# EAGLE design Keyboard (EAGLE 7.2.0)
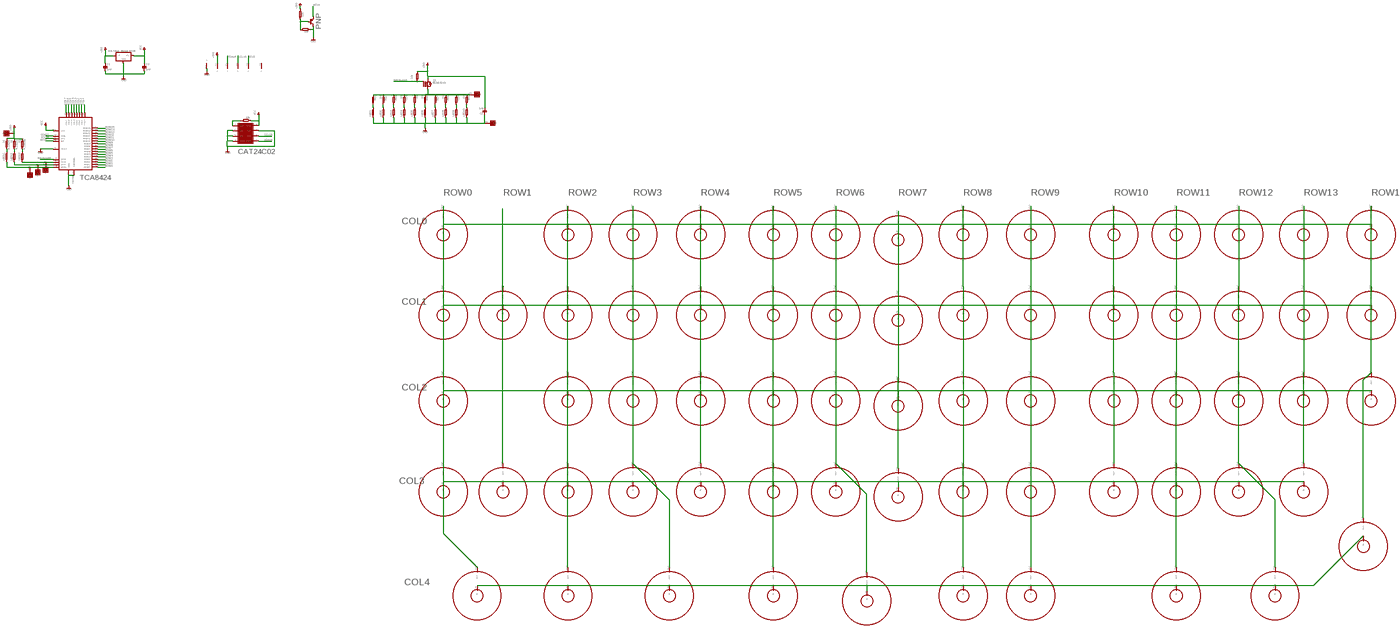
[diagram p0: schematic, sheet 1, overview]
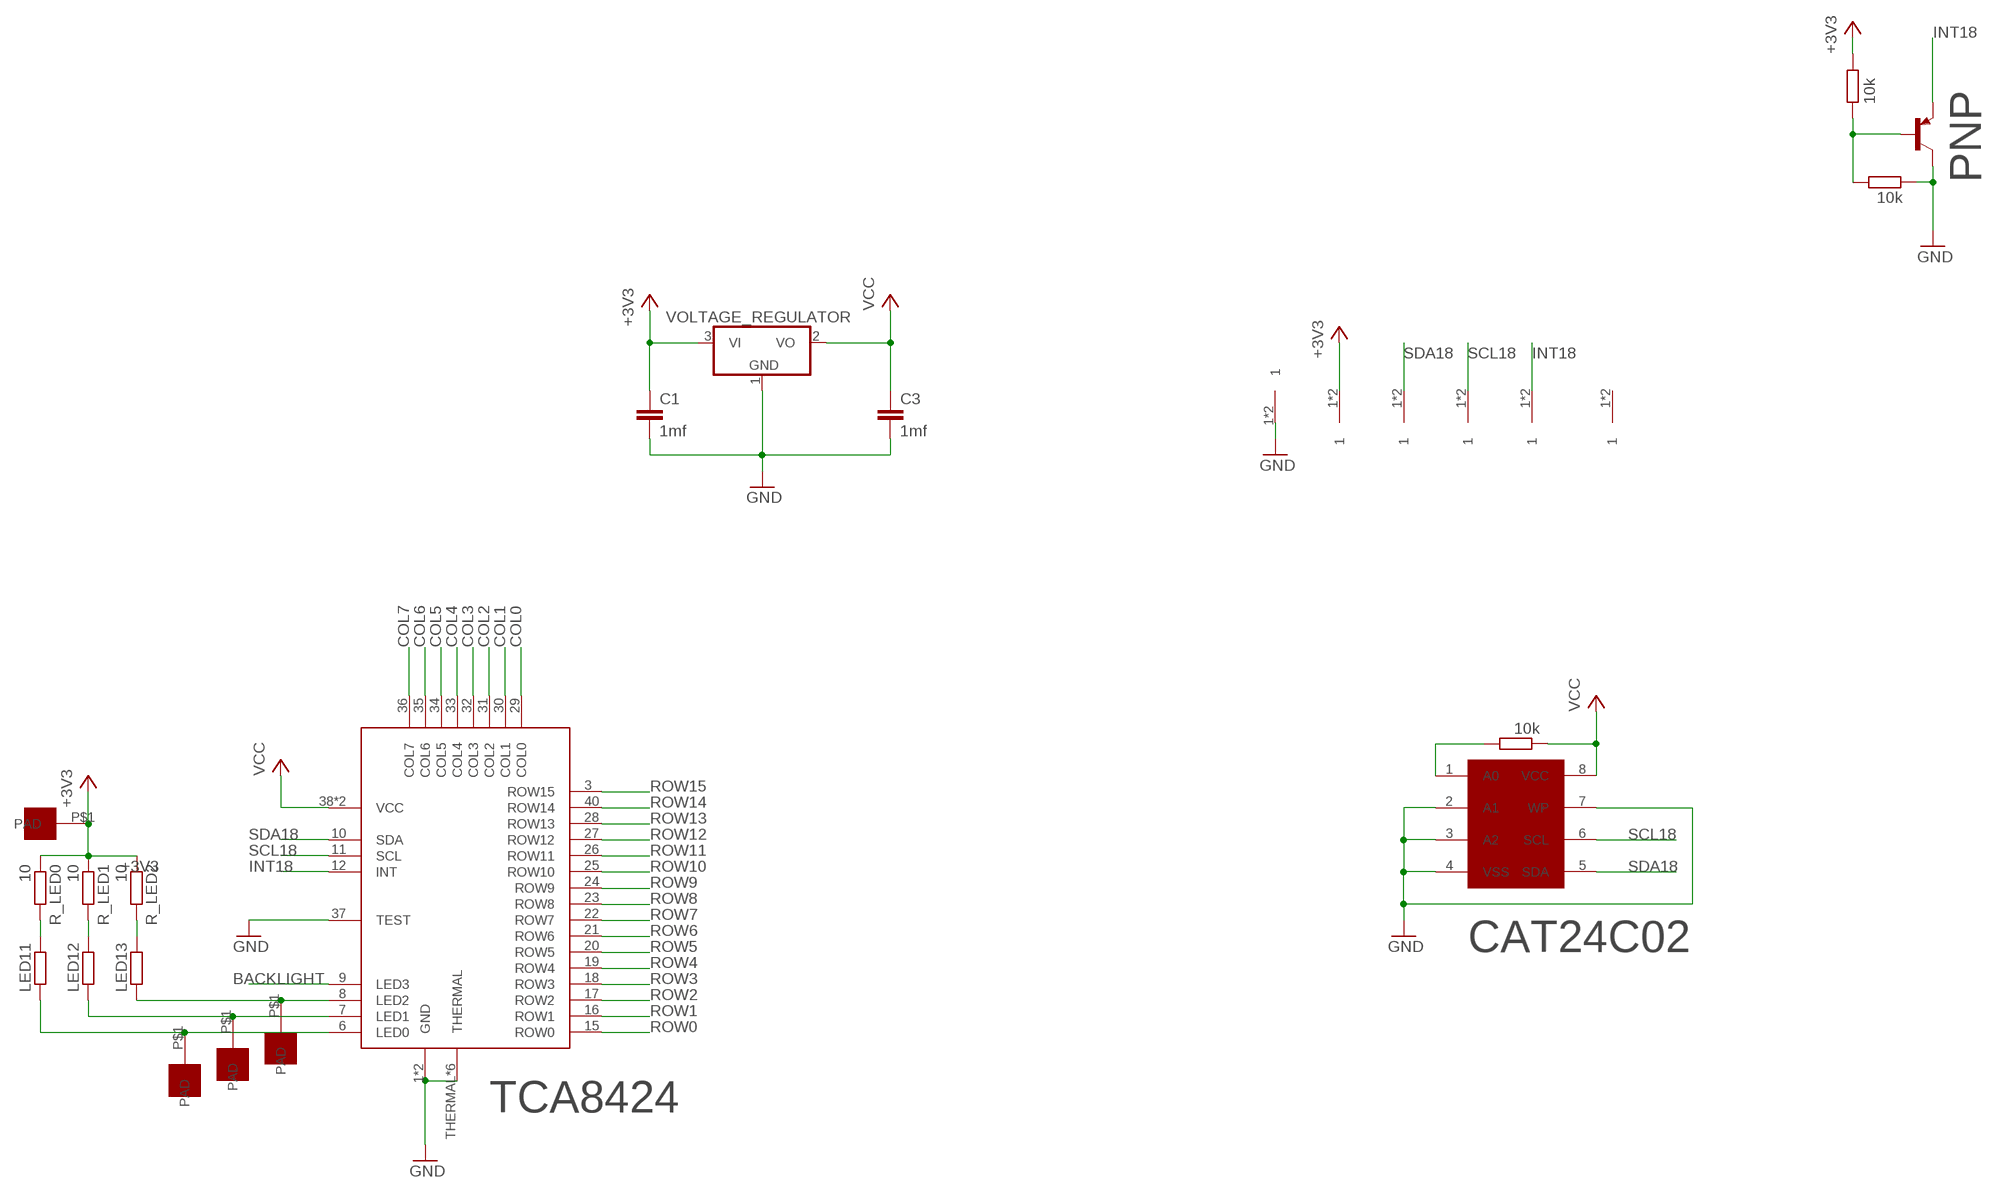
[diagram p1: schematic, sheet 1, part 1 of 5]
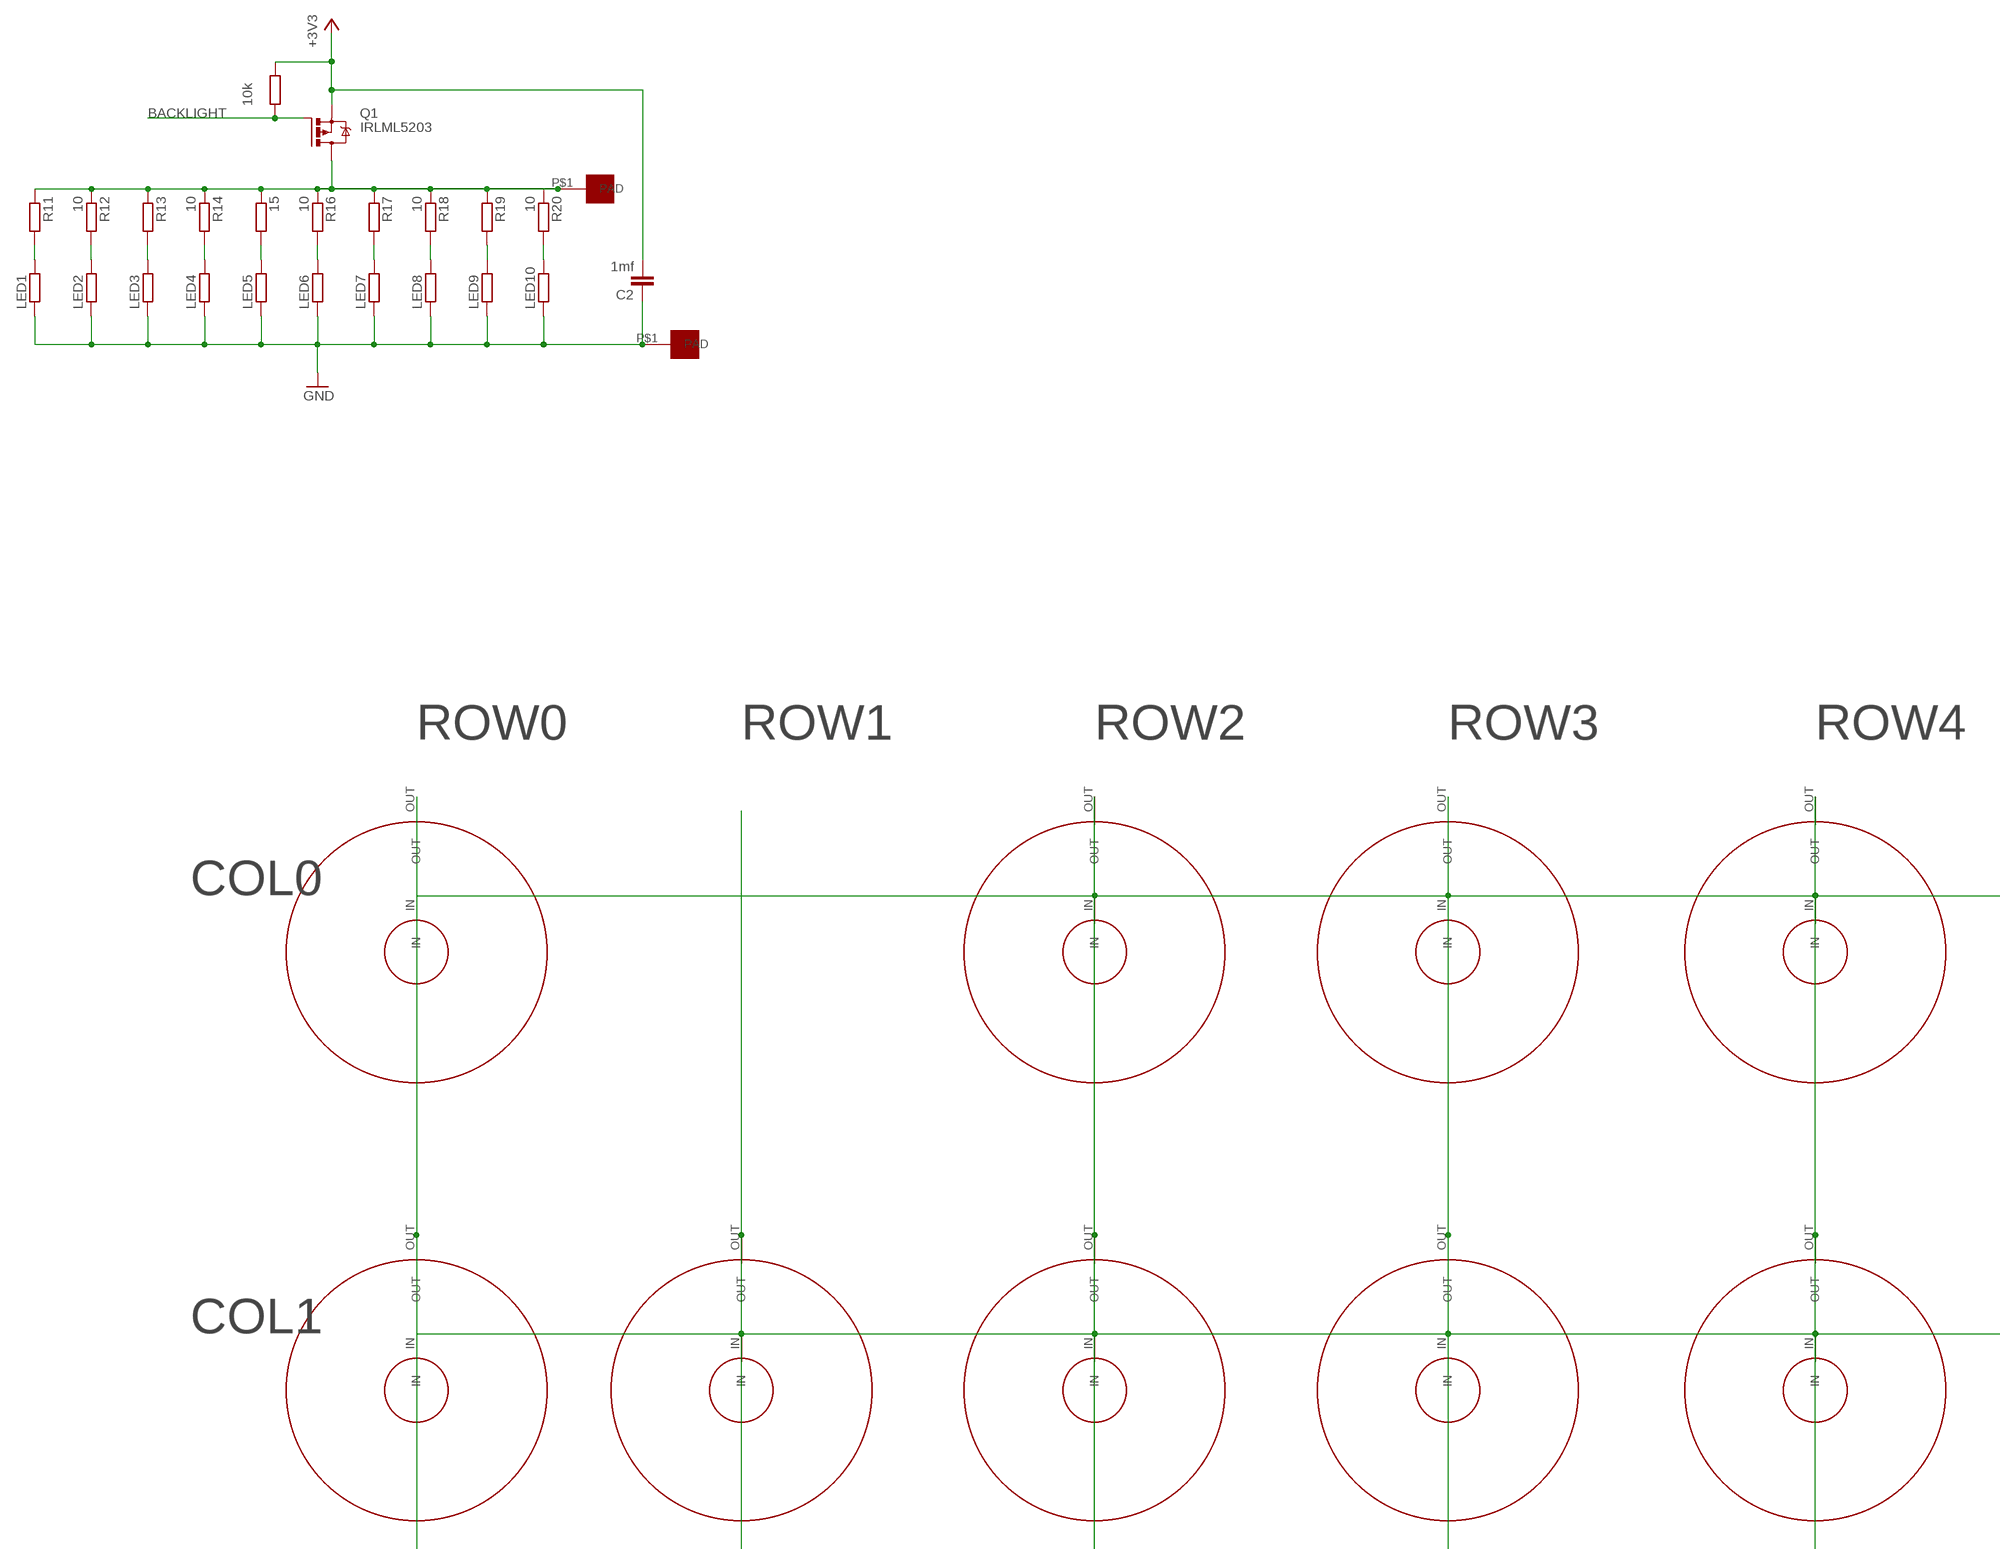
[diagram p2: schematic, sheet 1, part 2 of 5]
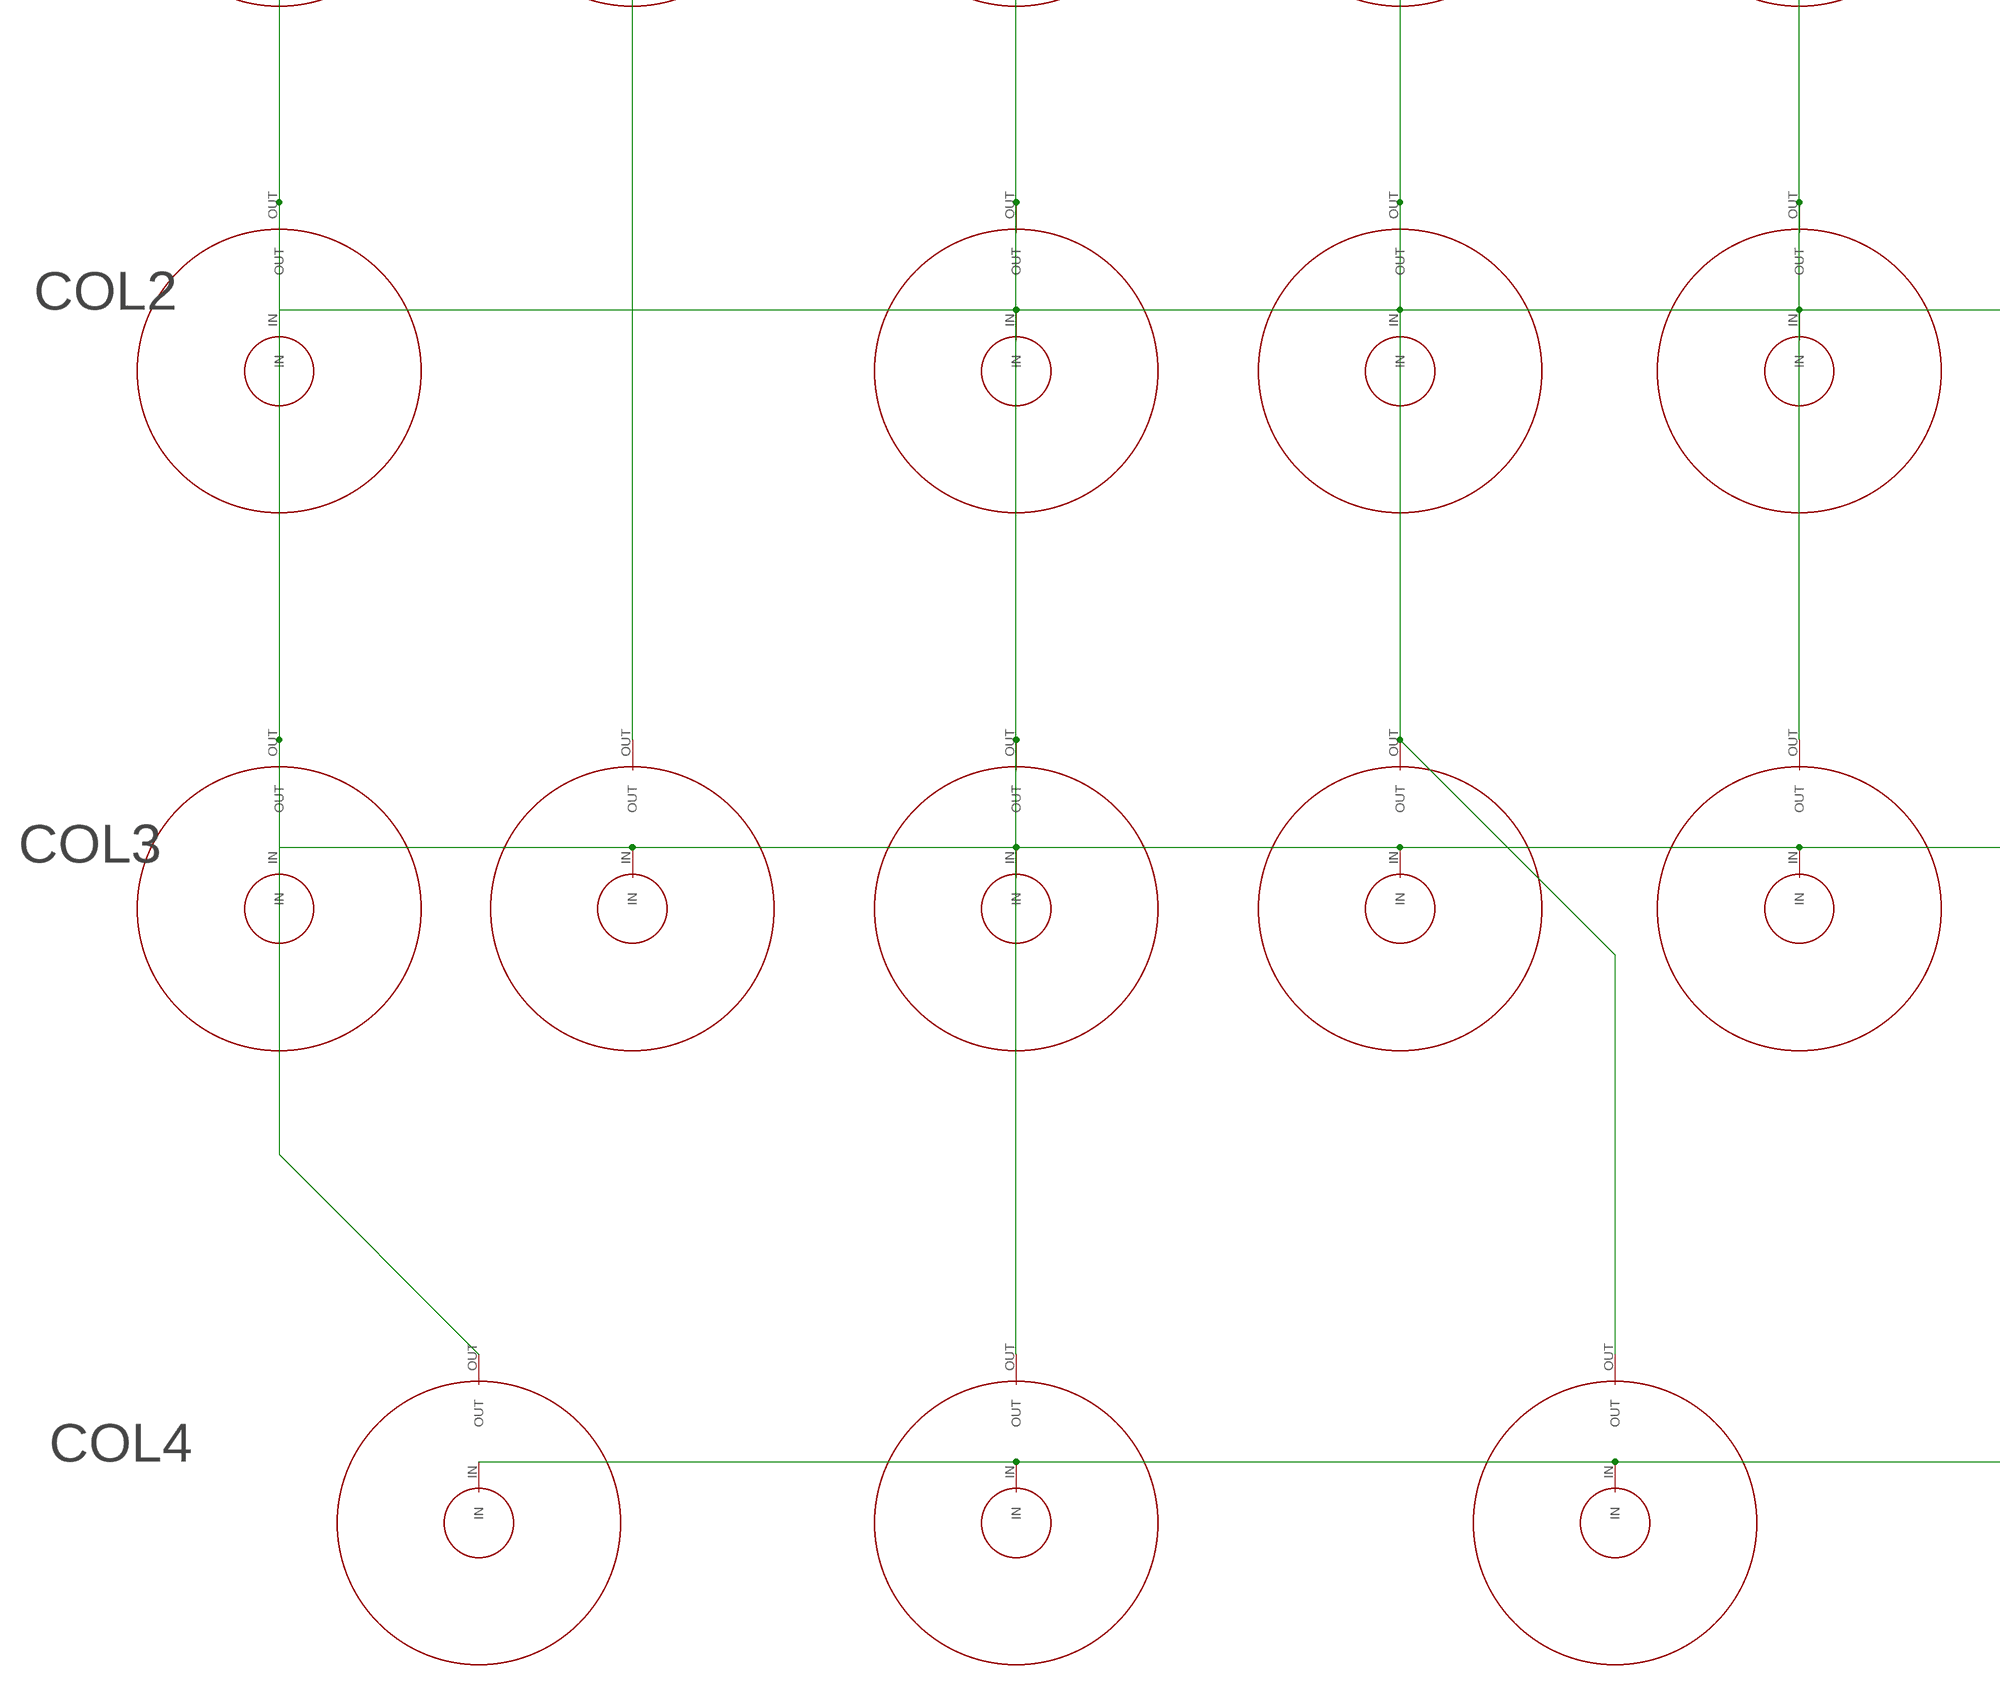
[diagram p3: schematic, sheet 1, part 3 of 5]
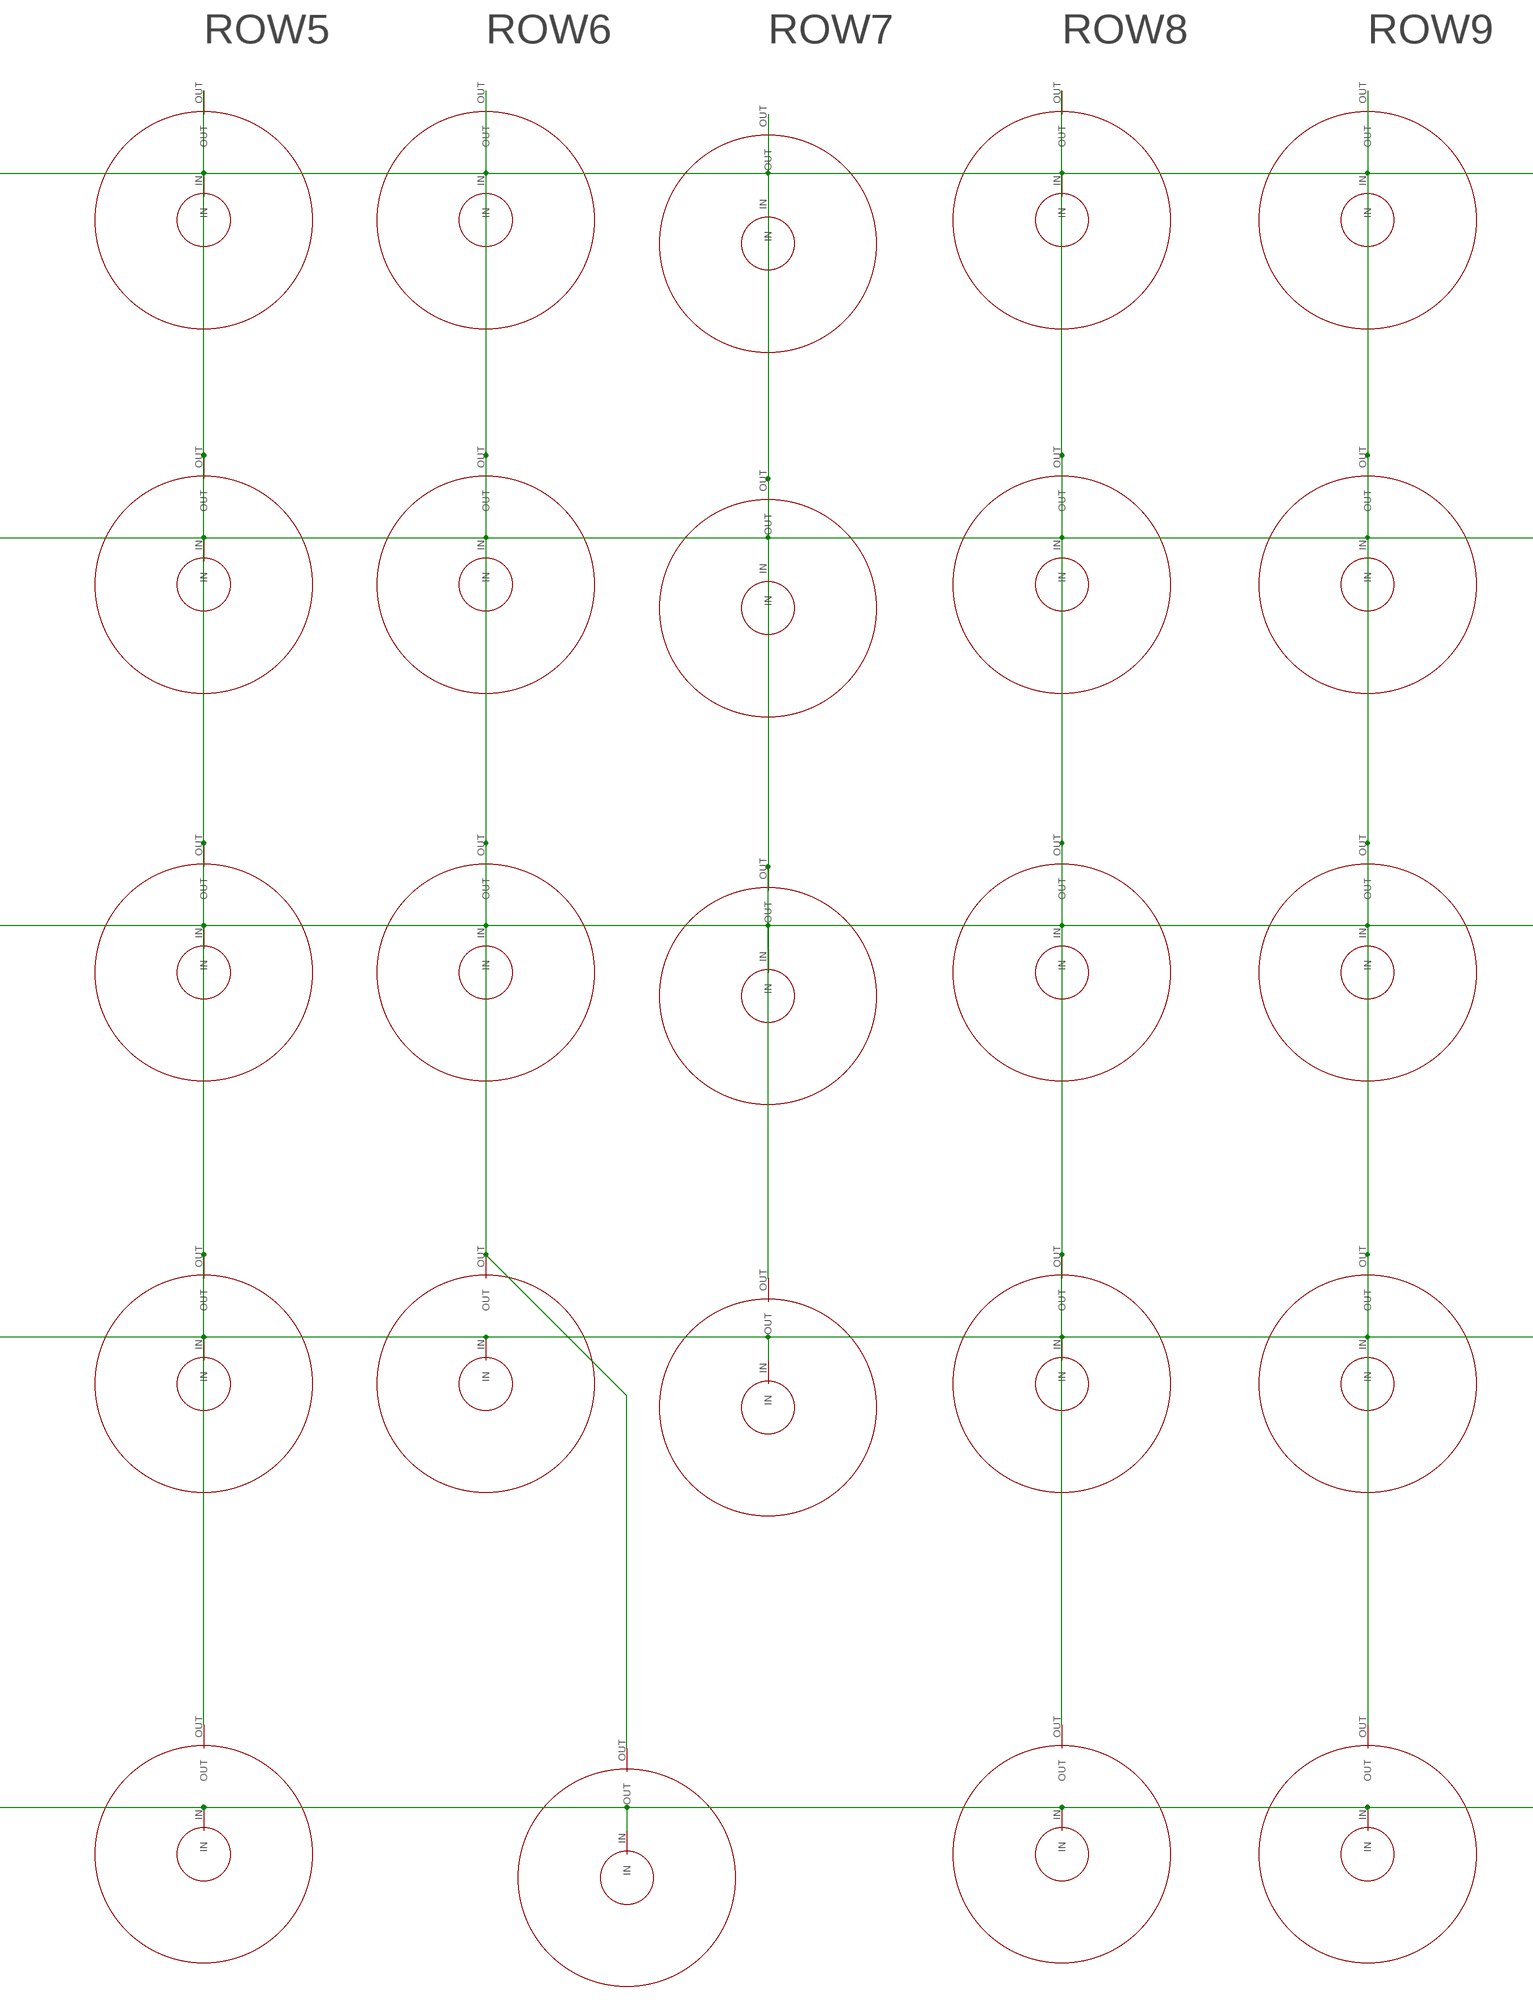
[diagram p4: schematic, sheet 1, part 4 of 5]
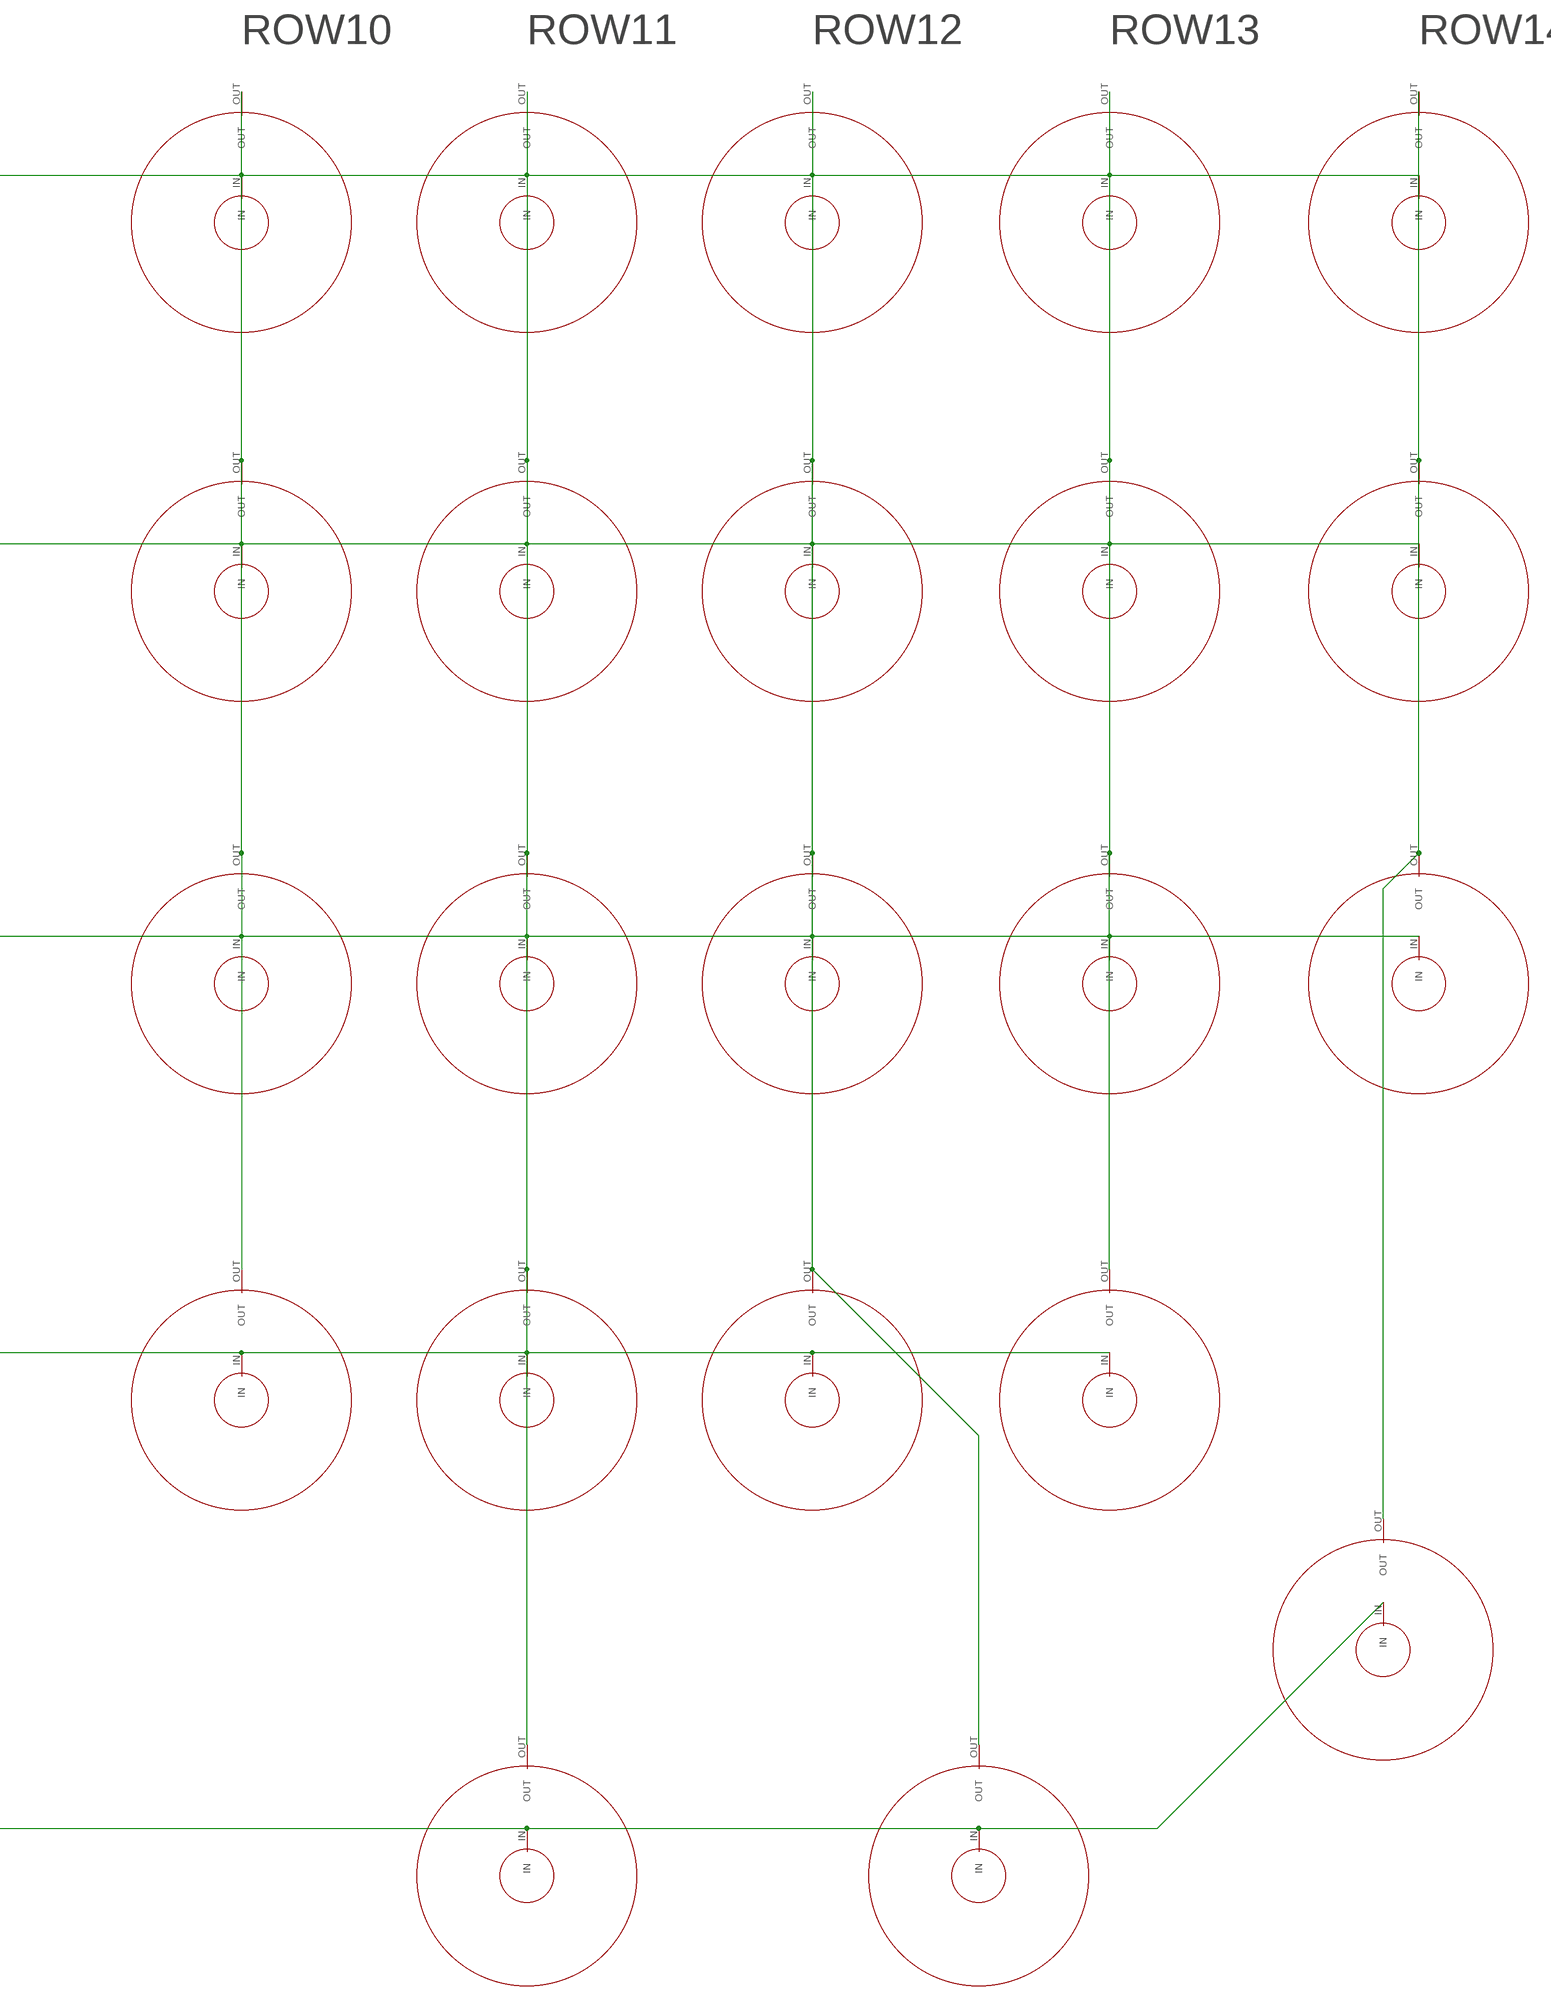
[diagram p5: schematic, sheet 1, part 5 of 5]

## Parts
15  R-EU_R0603  [R0603]
+  PAD  [PAD]
BL_PULLUP  10k  R-EU_R0603  [R0603]
C1  1mf  C-EUC0603  [C0603]
C2  1mf  C-EUC0603  [C0603]
C3  1mf  C-EUC0603  [C0603]
LED1  R-EU_R0402  [R0402]
LED2  R-EU_R0402  [R0402]
LED3  R-EU_R0402  [R0402]
LED4  R-EU_R0402  [R0402]
LED5  R-EU_R0402  [R0402]
LED6  R-EU_R0402  [R0402]
LED7  R-EU_R0402  [R0402]
LED8  R-EU_R0402  [R0402]
LED9  R-EU_R0402  [R0402]
LED10  R-EU_R0402  [R0402]
LED11  R-EU_R0402  [R0402]
LED12  R-EU_R0402  [R0402]
LED13  R-EU_R0402  [R0402]
PNP_DOWN  10k  R-EU_R0603  [R0603]
PNP_DOWN1  10k  R-EU_R0603  [R0603]
PNP_UP  10k  R-EU_R0603  [R0603]
Q1  IRLML5203  [MICRO3]
Q2  MMBTA56-SOT23  [SOT23]
R11  R-EU_R0603  [R0603]
R12  10  R-EU_R0603  [R0603]
R13  R-EU_R0603  [R0603]
R14  10  R-EU_R0603  [R0603]
R16  10  R-EU_R0603  [R0603]
R17  R-EU_R0603  [R0603]
R18  10  R-EU_R0603  [R0603]
R19  R-EU_R0603  [R0603]
R20  10  R-EU_R0603  [R0603]
R_LED0  10  R-EU_R0603  [R0603]
R_LED1  10  R-EU_R0603  [R0603]
R_LED2  10  R-EU_R0603  [R0603]
U$1  CAT24  [CAT24]
U$2  TCA8424  [QFN40]
U$3  BOTTOM_POGO  [POGO]
U$4  BOTTOM_POGO  [POGO]
U$5  BOTTOM_POGO  [POGO]
U$6  BOTTOM_POGO  [POGO]
U$7  BOTTOM_POGO  [POGO]
U$8  BOTTOM_POGO  [POGO]
U$9  DOME  [4MM]
U$11  DOME  [4MM]
U$12  DOME  [4MM]
U$13  DOME  [4MM]
U$14  DOME  [4MM]
U$15  DOME  [4MM]
U$16  DOME  [4MM]
U$17  DOME  [4MM]
U$18  DOME  [4MM]
U$19  DOME  [4MM]
U$20  DOME  [4MM]
U$21  DOME  [4MM]
U$22  DOME  [4MM]
U$23  DOME  [4MM]
U$24  DOME  [4MM]
U$25  DOME  [4MM]
U$26  DOME  [4MM]
U$27  DOME  [4MM]
U$28  DOME  [4MM]
U$29  DOME  [4MM]
U$30  DOME  [4MM]
U$31  DOME  [4MM]
U$32  DOME  [4MM]
U$33  DOME  [4MM]
U$34  DOME  [4MM]
U$35  DOME  [4MM]
U$36  DOME  [4MM]
U$37  DOME  [4MM]
U$38  DOME  [4MM]
U$39  DOME  [4MM]
U$40  DOME  [4MM]
U$41  DOME  [4MM]
U$42  DOME  [4MM]
U$43  DOME  [4MM]
U$44  DOME  [4MM]
U$45  DOME  [4MM]
U$46  DOME  [4MM]
U$47  DOME  [4MM]
U$48  DOME  [4MM]
U$49  DOME  [4MM]
U$50  DOME  [4MM]
U$51  DOME  [4MM]
U$52  DOME  [4MM]
U$53  PAD  [PAD]
U$54  DOME  [4MM]
U$55  DOME  [4MM]
U$56  DOME  [4MM]
U$57  DOME  [4MM]
U$58  DOME  [4MM]
U$59  DOME  [4MM]
U$60  DOME  [4MM]
U$61  DOME  [4MM]
U$62  DOME  [4MM]
U$63  DOME  [4MM]
U$64  DOME  [4MM]
U$65  DOME  [4MM]
U$66  DOME  [4MM]
U$67  DOME  [4MM]
U$68  DOME  [4MM]
U$69  DOME  [4MM]
U$70  DOME  [4MM]
U$71  PAD  [PAD]
U$72  DOME  [4MM]
U$73  DOME  [4MM]
U$74  PAD  [PAD]
U$75  DOME  [4MM]
U$76  DOME  [4MM]
U$77  DOME  [4MM]
U$78  PAD  [PAD]
U$79  DOME  [4MM]
U$80  PAD  [PAD]
U$81  DOME  [4MM]
VOLTAGE_REGULATOR  MCP1703CB  [SOT23]

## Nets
+3V3: +.P$1(PAD) BL_PULLUP.1 C1.1 C2.2 PNP_UP.1 Q1.2(S) R_LED0.1 R_LED1.1 R_LED2.1 U$4.1 U$4.P$2 VOLTAGE_REGULATOR.3(VI)
BACKLIGHT: BL_PULLUP.2 Q1.1(G) U$2.9(LED3)
COL0: U$2.29(COL0) U$9.IN U$11.IN U$12.IN U$13.IN U$14.IN U$15.IN U$16.IN U$17.IN U$18.IN U$19.IN U$20.IN U$21.IN U$22.IN U$23.IN
COL1: U$2.30(COL1) U$24.IN U$25.IN U$26.IN U$27.IN U$28.IN U$29.IN U$30.IN U$31.IN U$32.IN U$33.IN U$34.IN U$35.IN U$36.IN U$37.IN U$38.IN
COL2: U$2.31(COL2) U$39.IN U$40.IN U$41.IN U$42.IN U$43.IN U$44.IN U$45.IN U$46.IN U$47.IN U$48.IN U$49.IN U$50.IN U$51.IN U$52.IN
COL3: U$2.32(COL3) U$54.IN U$55.IN U$56.IN U$57.IN U$58.IN U$59.IN U$60.IN U$61.IN U$62.IN U$63.IN U$64.IN U$65.IN U$66.IN U$68.IN
COL4: U$2.33(COL4) U$67.IN U$69.IN U$70.IN U$72.IN U$73.IN U$75.IN U$76.IN U$77.IN U$79.IN U$81.IN
COL5: U$2.34(COL5)
COL6: U$2.35(COL6)
COL7: U$2.36(COL7)
DRAIN: 15.1 Q1.3(D) R11.1 R12.1 R13.1 R14.1 R16.1 R17.1 R18.1 R19.1 R20.1 U$78.P$1(PAD)
GND: C1.2 C2.1 C3.2 LED1.1 LED2.1 LED3.1 LED4.1 LED5.1 LED6.1 LED7.1 LED8.1 LED9.1 LED10.1 PNP_DOWN.2 Q2.3(C) U$1.2(A1) U$1.3(A2) U$1.4(VSS) U$1.7(WP) U$2.1(GND) U$2.4(GND) U$2.37(TEST) U$2.THERMAL U$2.VIA1(THERMAL) U$2.VIA2(THERMAL) U$2.VIA3(THERMAL) U$2.VIA4(THERMAL) U$2.VIA5(THERMAL) U$3.1 U$3.P$2 U$80.P$1(PAD) VOLTAGE_REGULATOR.1(GND)
INT18: Q2.2(E) U$2.12(INT) U$7.1 U$7.P$2
LED_GROUND0: LED11.2 R_LED0.2
LED_GROUND1: LED12.2 R_LED1.2
LED_GROUND2: LED13.2 R_LED2.2
N$1: LED1.2 R11.2
N$2: LED2.2 R12.2
N$3: LED3.2 R13.2
N$4: LED4.2 R14.2
N$6: 15.2 LED5.2
N$7: LED6.2 R16.2
N$8: LED7.2 R17.2
N$9: LED8.2 R18.2
N$10: LED9.2 R19.2
N$11: LED10.2 R20.2
N$13: PNP_DOWN.1 PNP_UP.2 Q2.1(B)
N$14: LED12.1 U$2.7(LED1) U$71.P$1(PAD)
N$15: LED11.1 U$2.6(LED0) U$53.P$1(PAD)
N$16: LED13.1 U$2.8(LED2) U$74.P$1(PAD)
N$17: PNP_DOWN1.2 U$1.1(A0)
ROW0: U$2.15(ROW0) U$9.OUT U$24.OUT U$39.OUT U$54.OUT U$69.OUT
ROW1: U$2.16(ROW1) U$38.OUT U$68.OUT
ROW2: U$2.17(ROW2) U$11.OUT U$25.OUT U$40.OUT U$55.OUT U$70.OUT
ROW3: U$2.18(ROW3) U$12.OUT U$26.OUT U$41.OUT U$56.OUT U$72.OUT
ROW4: U$2.19(ROW4) U$13.OUT U$27.OUT U$42.OUT U$57.OUT
ROW5: U$2.20(ROW5) U$14.OUT U$28.OUT U$43.OUT U$58.OUT U$73.OUT
ROW6: U$2.21(ROW6) U$15.OUT U$29.OUT U$44.OUT U$59.OUT U$75.OUT
ROW7: U$2.22(ROW7) U$16.OUT U$30.OUT U$45.OUT U$60.OUT
ROW8: U$2.23(ROW8) U$17.OUT U$31.OUT U$46.OUT U$61.OUT U$76.OUT
ROW9: U$2.24(ROW9) U$18.OUT U$32.OUT U$47.OUT U$62.OUT U$77.OUT
ROW10: U$2.25(ROW10) U$19.OUT U$33.OUT U$48.OUT U$63.OUT
ROW11: U$2.26(ROW11) U$20.OUT U$34.OUT U$49.OUT U$64.OUT U$79.OUT
ROW12: U$2.27(ROW12) U$21.OUT U$35.OUT U$50.OUT U$65.OUT U$81.OUT
ROW13: U$2.28(ROW13) U$22.OUT U$36.OUT U$51.OUT U$66.OUT
ROW14: U$2.40(ROW14) U$23.OUT U$37.OUT U$52.OUT U$67.OUT
ROW15: U$2.3(ROW15)
SCL18: U$1.6(SCL) U$2.11(SCL) U$6.1 U$6.P$2
SDA18: U$1.5(SDA) U$2.10(SDA) U$5.1 U$5.P$2
VCC: C3.1 PNP_DOWN1.1 U$1.8(VCC) U$2.38(VCC) U$2.39(VCC) VOLTAGE_REGULATOR.2(VO)
Unconnected: U$8.1 U$8.P$2

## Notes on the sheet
- PNP
- CAT24C02
- TCA8424

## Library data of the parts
15 BL_PULLUP LED1-LED13 PNP_DOWN PNP_DOWN1 PNP_UP R11-R14 R16-R20 R_LED0 R_LED1 R_LED2 = rcl:R-EU_: RESISTOR, European symbol
+ U$53 U$71 U$74 U$78 U$80 = PAD:PAD
C1-C3 = rcl:C-EU: CAPACITOR, European symbol
Q1 = transistor-power:IRLML5203: HEXFET P-Channel Power MOSFET
Q2 = transistor-pnp:*-?: PNP Transistor
U$1 = cat24:CAT24
U$2 = TCA8424:TCA8424
U$3-U$8 = bottom_pogo:BOTTOM_POGO
U$9 U$11-U$52 U$54-U$70 U$72 U$73 U$75-U$77 U$79 U$81 = DOME:DOME
VOLTAGE_REGULATOR = linear:MCP1703: 250 mA, 16V, Low Quiescent Current LDO Regulator Source: http://ww1.microchip.com/downloads/en/DeviceDoc/22049b.pdf

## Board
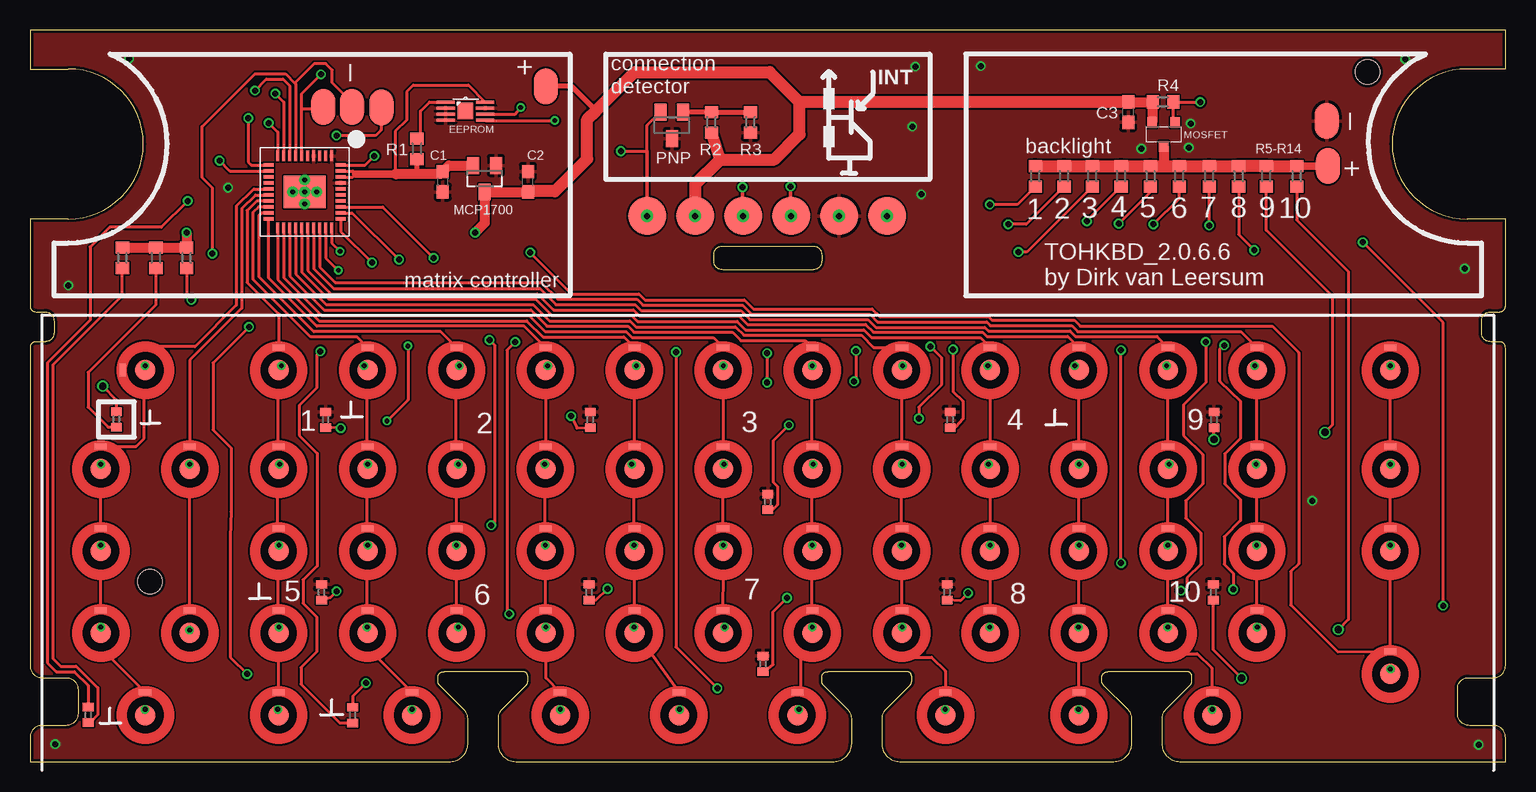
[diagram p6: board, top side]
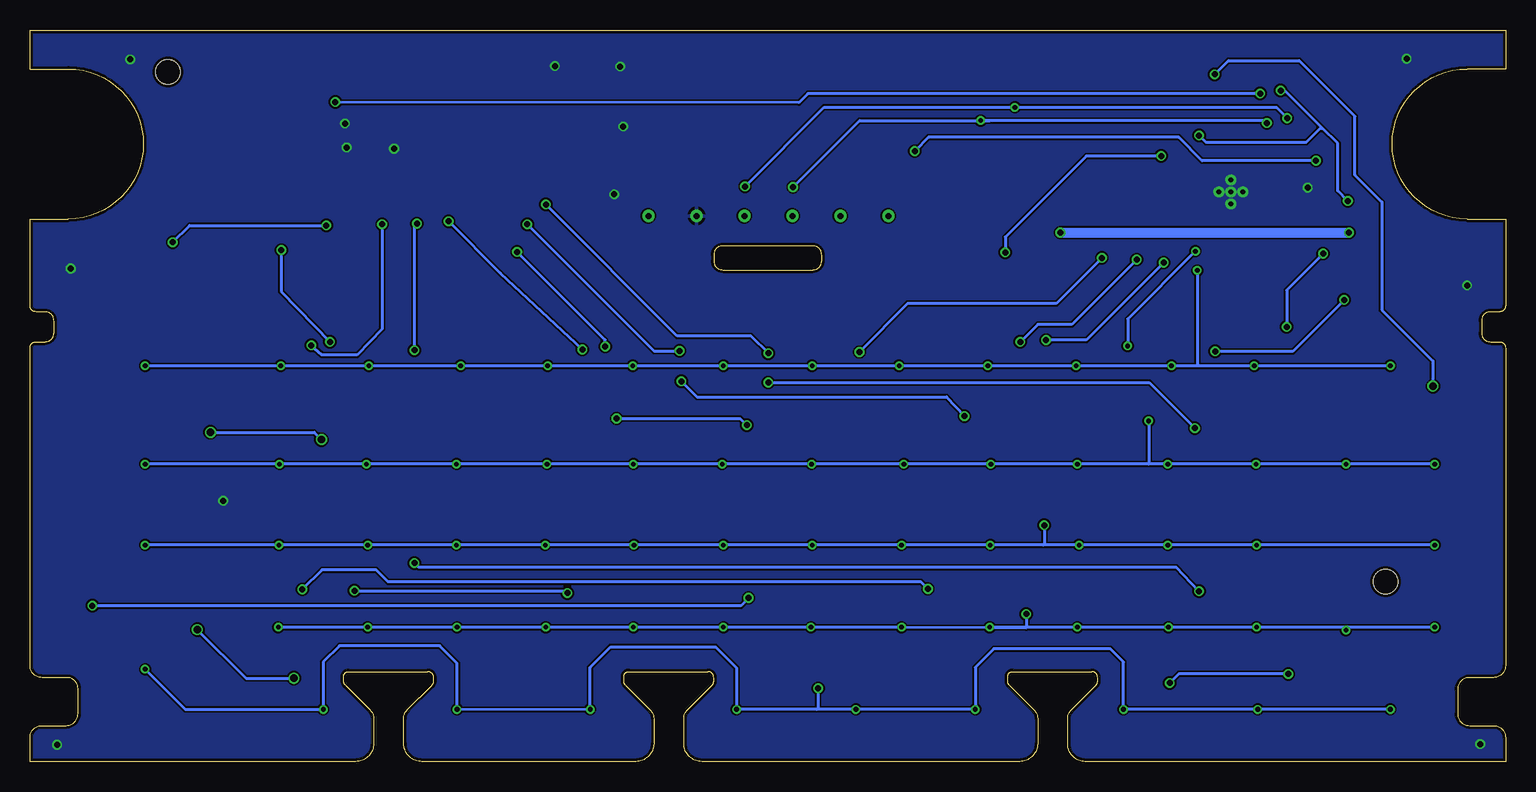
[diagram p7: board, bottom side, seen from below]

Size 123 x 61 mm. Coordinates in mm from the lower left corner, seen from the top.
Outline: 100 segments
Copper layers (1*16): Top 0.035mm / dielectric 1.5mm / Bottom 0.035mm
Design rules "ITEADstudio_DRC": minimum track width 6mil, minimum drill 12mil, track to track 6mil, track to pad 6mil, pad to pad 6mil, via to via 6mil, smd to smd 0mil, copper to edge 10mil, drill to drill 10mil, minimum pad ring 10mil, minimum via ring 6mil, stop-mask expansion 2mil, vias tented up to drill 100mil, thermal gap 10mil
Holes 2 mm at 10,15 111.5,57.5

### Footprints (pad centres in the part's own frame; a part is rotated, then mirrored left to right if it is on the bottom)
R0603 = smd 1 x 1.1: 1 -0.85,0; 2 0.85,0
PAD = smd 2 x 3: P$1 0,0
C0603 = smd 1.1 x 1: 1 -0.85,0; 2 0.85,0
R0402 = smd 0.7 x 0.9: 1 -0.65,0; 2 0.65,0
MICRO3 = smd 0.8 x 0.9: 1 -0.95,-1; 2 0.95,-1; 3 0,1
SOT23 = smd 1 x 1.4: 1 -0.95,-1.1; 2 0.95,-1.1; 3 0,1.1
CAT24 = smd 0.25 x 1.5: 1 -0.75,-1.65; 2 -0.25,-1.65; 3 0.25,-1.65; 4 0.75,-1.65; 5 0.75,1.65; 6 0.25,1.65; 7 -0.25,1.65; 8 -0.75,1.65 | smd 1.4 x 1.3: P$1 0,0
QFN40 = smd 0.85 x 0.28: 1 -3,2.25; 2 -3,1.75; 3 -3,1.25; 4 -3,0.75; 5 -3,0.25; 6 -3,-0.25; 7 -3,-0.75; 8 -3,-1.25; 9 -3,-1.75; 10 -3,-2.25; 21 3,-2.25; 22 3,-1.75; 23 3,-1.25; 24 3,-0.75; 25 3,-0.25; 26 3,0.25; 27 3,0.75; 28 3,1.25; 29 3,1.75; 30 3,2.25 | smd 0.28 x 0.85: 11 -2.25,-3; 12 -1.75,-3; 13 -1.25,-3; 14 -0.75,-3; 15 -0.25,-3; 16 0.25,-3; 17 0.75,-3; 18 1.25,-3; 19 1.75,-3; 20 2.25,-3; 31 2.25,3; 32 1.75,3; 33 1.25,3; 34 0.75,3; 35 0.25,3; 36 -0.25,3; 37 -0.75,3; 38 -1.25,3; 39 -1.75,3; 40 -2.25,3 | smd 2.7 x 3.5: P$2 0,0 | smd 1 x 1.5: P$11 -0.65,0.9; P$12 0.65,0.9; P$13 0.65,-0.9; THERMAL -0.65,-0.9 | drill 0.4 pad 0.406: VIA1 0,1; VIA2 -1,0; VIA3 0,0; VIA4 1,0; VIA5 0,-1
POGO = smd 3.175 x 3.175: 1 0,0 | drill 0.5: P$2 0,0
4MM = smd 1.7 x 1.7: IN 0,0 | smd 1 x 0.5: OUT 0,1.9

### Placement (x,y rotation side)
15  93.4,48.8 270 top
+  43,56.3 0 top
BL_PULLUP  94.45,55 0 top
C1  41.5,48.35 90 top
C2  91.55,54.15 90 top
C3  34.4,48.35 270 top
LED1  24.65,28.5 270 top
LED2  46.7,28.5 270 top
LED3  61.5,21.65 270 top
LED4  76.7,28.5 270 top
LED5  24.3,14.12 270 top
LED6  46.6,14.12 270 top
LED7  61.1,8.15 270 top
LED8  98.7,28.5 270 top
LED9  76.45,14.12 270 top
LED10  98.65,14.12 270 top
LED11  7.2,28.53 270 top
LED12  26.9,3.87 270 top
LED13  4.85,3.9 270 top
PNP_DOWN  60.05,53.3 270 top
PNP_DOWN1  32.25,51.1 90 top
PNP_UP  56.8,53.3 90 top
Q1  94.5,52.3 180 top
Q2  53.5,53.05 180 top
R11  83.8,48.8 270 top
R12  86.2,48.8 270 top
R13  88.55,48.8 270 top
R14  90.95,48.8 270 top
R16  95.8,48.8 270 top
R17  98.3,48.8 270 top
R18  103.05,48.8 270 top
R19  100.75,48.8 270 top
R20  105.6,48.8 270 top
R_LED0  10.5,42 270 top
R_LED1  13.05,42 270 top
R_LED2  7.7,42 270 top
U$1  36.3,54.25 270 top
U$2  22.9,47.5 270 top
U$3  67.45,45.5 90 top
U$4  55.45,45.5 90 top
U$5  59.45,45.5 90 top
U$6  63.45,45.5 90 top
U$7  51.45,45.5 90 top
U$8  71.45,45.5 0 top
U$9  9.61,32.63 90 top
U$11  20.73,32.63 0 top
U$12  28.14,32.63 0 top
U$13  35.56,32.63 0 top
U$14  42.97,32.63 0 top
U$15  50.38,32.63 0 top
U$16  57.79,32.63 0 top
U$17  65.21,32.63 0 top
U$18  72.67,32.63 0 top
U$19  80.03,32.63 0 top
U$20  87.44,32.63 0 top
U$21  94.86,32.63 0 top
U$22  102.27,32.63 0 top
U$23  113.39,32.63 0 top
U$24  5.91,24.39 0 top
U$25  20.73,24.39 0 top
U$26  28.14,24.39 0 top
U$27  35.56,24.39 0 top
U$28  42.97,24.39 0 top
U$29  50.38,24.39 0 top
U$30  57.79,24.39 0 top
U$31  65.21,24.39 0 top
U$32  72.67,24.39 0 top
U$33  80.03,24.39 0 top
U$34  87.44,24.39 0 top
U$35  94.86,24.39 0 top
U$36  102.27,24.39 0 top
U$37  113.39,24.39 0 top
U$38  13.32,24.39 0 top
U$39  5.91,17.55 0 top
U$40  20.73,17.55 0 top
U$41  28.14,17.55 0 top
U$42  35.56,17.55 0 top
U$43  42.97,17.55 0 top
U$44  50.38,17.55 0 top
U$45  57.79,17.55 0 top
U$46  65.21,17.55 0 top
U$47  72.67,17.55 0 top
U$48  80.03,17.55 0 top
U$49  87.44,17.55 0 top
U$50  94.86,17.55 0 top
U$51  102.27,17.55 0 top
U$52  113.39,17.55 0 top
U$53  24.45,54.6 0 top
U$54  5.91,10.71 0 top
U$55  20.73,10.71 0 top
U$56  28.14,10.71 0 top
U$57  35.56,10.71 0 top
U$58  42.97,10.71 0 top
U$59  50.38,10.71 0 top
U$60  57.79,10.71 0 top
U$61  65.21,10.71 0 top
U$62  72.67,10.71 0 top
U$63  80.03,10.71 0 top
U$64  87.44,10.71 0 top
U$65  94.86,10.71 0 top
U$66  102.27,10.71 0 top
U$67  113.39,7.3 0 top
U$68  13.32,10.71 0 top
U$69  9.61,3.87 0 top
U$70  20.73,3.87 0 top
U$71  26.85,54.6 0 top
U$72  31.85,3.87 0 top
U$73  44.2,3.87 0 top
U$74  29.3,54.55 0 top
U$75  54.09,3.87 0 top
U$76  63.97,3.87 0 top
U$77  76.33,3.87 0 top
U$78  108.2,49.65 0 top
U$79  87.44,3.87 0 top
U$80  108.1,53.4 0 top
U$81  98.56,3.87 0 top
VOLTAGE_REGULATOR  37.9,48.6 180 top

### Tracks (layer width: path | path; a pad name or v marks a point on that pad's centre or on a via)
+3V3  (via drill 0.5)
  Top 0.254: PNP_UP.1 56.85,52.25 | C1.1 41.55,47.55
  Top 0.406: 47.17,54.27 45.15,56.3 +.P$1
  Top 0.813: C1.1 VOLTAGE_REGULATOR.3 37.9,44.9 v37.1,44.1 | v13.05,44.1 13.05,42.95 | 13.05,42.95 12.7,42.85 R_LED0.1 R_LED2.1 | R_LED1.1 13.05,42.95 | C2.2 BL_PULLUP.1 93.55,55 Q1.2
  Top 1.016: C2.2 64.15,55 | 41.55,47.55 43.75,47.55 46.45,50.25 46.45,53.55 47.17,54.27 50.4,57.5 61.65,57.5 64.15,55 | 57.5,50.2 55.45,48.15 U$4.P$2 | 57.5,50.2 62.05,50.2 64.15,52.3 64.15,55 | 56.85,52.25 57.5,50.2
  Bottom 0.813: v37.1,44.1 v13.05,44.1
BACKLIGHT  (via drill 0.5)
  Top 0.254: v20.45,55.7 21.15,55 U$2.9 | Q1.1 95.3,53.3 BL_PULLUP.2 v97.55,55
  Bottom 0.254: v20.45,55.7 58.15,55.7 58.9,54.95 v97.55,55
COL0  (via drill 0.4)
  Top 0.254: v113.4,33 arc-183 U$23.IN | U$22.IN 102.1,32.8 v102.1,33 | U$21.IN 94.75,32.74 v94.75,33 | U$20.IN 87.1,32.97 v87.1,33 | U$19.IN 79.85,32.81 v79.85,33 | U$18.IN 72.75,32.71 v72.75,33 | U$17.IN 64.84,33 v65.2,33 | U$16.IN 57.42,33 v57.8,33 | U$15.IN 50.55,32.8 v50.55,33 | U$14.IN 43.15,32.81 v43.15,33 | U$13.IN 35.8,32.87 v35.8,33 | U$12.IN 27.85,32.92 v27.85,33 | U$11.IN 20.85,32.75 | 20.85,32.75 20.85,33 | 20.85,32.75 20.95,32.85 v20.95,33 | U$2.29 24.65,42 v25.7,40.95
  Top 0.406: U$9.IN v9.6,33
  Bottom 0.254: v9.6,33 v20.95,33 25.8,33 | 25.8,33 v27.85,33 v35.8,33 v43.15,33 v50.55,33 v57.8,33 | v57.8,33 v65.2,33 v72.75,33 v79.85,33 v87.1,33 v94.75,33 v102.1,33 v113.4,33 | v57.8,33 57.55,33 | v25.7,40.95 25.7,33.1 25.8,33
COL1  (via drill 0.4)
  Top 0.254: U$24.IN v5.9,24.8 | v113.4,24.8 U$37.IN | U$38.IN arc-90 13.3,24.41 v13.3,24.8 | U$25.IN arc90 20.8,24.46 v20.8,24.8 | U$26.IN arc90 28.45,24.7 v28.15,24.8 | U$27.IN arc90 35.7,24.53 v35.7,24.8 | U$28.IN arc-90 42.95,24.41 42.95,24.8 v42.9,24.8 | U$29.IN arc-90 50.15,24.62 v50.15,24.8 | U$30.IN arc90 57.85,24.45 v57.85,24.8 | U$31.IN arc90 65.3,24.48 v65.3,24.8 | U$32.IN arc90 72.7,24.42 v72.7,24.8 | U$33.IN arc-90 79.9,24.52 v79.9,24.8 | U$34.IN arc-90 87.15,24.68 v87.45,24.8 | U$35.IN arc90 94.95,24.48 v94.95,24.8 | U$36.IN arc-90 102.2,24.46 v102.2,24.8 | U$2.30 25.15,43.25 v25.85,42.55 | v31.5,34.65 31.5,30.15 v29.75,28.4
  Bottom 0.254: v5.9,24.8 v13.3,24.8 v20.8,24.8 v28.15,24.8 29.75,24.8 | 29.75,24.8 v35.7,24.8 v42.9,24.8 v50.15,24.8 v57.85,24.8 v65.3,24.8 v72.7,24.8 v79.9,24.8 v87.45,24.8 v94.95,24.8 v102.2,24.8 v113.4,24.8 | v25.85,42.55 31.5,36.9 v31.5,34.65 | v29.75,28.4 29.75,24.8
COL2  (via drill 0.4, 0.5)
  Top 0.254: U$39.IN v5.9,18.05 | v113.4,18.05 U$52.IN | U$51.IN 102.27,18.03 v102.25,18.05 | U$50.IN v94.86,18.04 v94.85,18.05 | U$49.IN v87.44,18.04 v87.45,18.05 | U$48.IN 80.03,18.03 v80.05,18.05 | U$47.IN 72.67,18.03 v72.65,18.05 | U$46.IN v65.21,18.04 v65.2,18.05 | U$45.IN v57.79,18.04 v57.8,18.05 | U$44.IN 50.38,18.02 v50.35,18.05 | U$43.IN 42.97,18.03 v42.95,18.05 | U$42.IN v35.56,18.04 v35.55,18.05 | U$41.IN 28.14,17.94 v28.15,18.05 | U$40.IN 20.63,17.83 v20.75,18.05 | U$2.31 25.9,44.2 v28.5,41.6 | v38.45,19.7 38.75,20 38.75,34.7 v38.3,35.15
  Bottom 0.254: v5.9,18.05 v20.75,18.05 v28.15,18.05 v35.55,18.05 38.55,18.05 | 38.55,18.05 v42.95,18.05 v50.35,18.05 v57.8,18.05 v65.2,18.05 v72.65,18.05 v80.05,18.05 v87.45,18.05 v94.85,18.05 v102.25,18.05 v113.4,18.05 | v38.45,19.7 38.45,18.15 38.55,18.05 | v28.5,41.6 34.95,35.15 v38.3,35.15
COL3  (via drill 0.4, 0.5)
  Top 0.254: U$54.IN v5.9,11.2 | v102.3,11.2 102.27,11.25 U$66.IN | U$55.IN 20.75,10.71 v20.75,11.2 | U$56.IN 28.1,10.71 v28.1,11.2 | U$57.IN 35.7,10.71 v35.7,11.2 | U$58.IN 43,10.71 v43,11.2 | U$59.IN 50.15,10.71 v50.35,11.2 | U$60.IN 57.9,10.71 v57.9,11.2 | U$61.IN v65.2,11.2 | U$62.IN 72.7,10.71 v72.7,11.2 | U$63.IN 80,10.71 v80,11.2 | U$64.IN 87.4,10.71 v87.4,11.2 | U$65.IN v94.85,11.2 | U$68.IN v13.3,10.95 | U$2.32 26.85,45.75 v30.75,41.85 | v40.45,35 39.75,34.3 39.75,12.5 v39.95,12.3
  Bottom 0.254: v5.9,11.2 13.3,11.2 | 13.3,11.2 v20.75,11.2 v28.1,11.2 v35.7,11.2 v43,11.2 39.95,11.15 | 39.95,11.15 v50.35,11.2 v57.9,11.2 v65.2,11.2 v72.7,11.2 v80,11.2 v87.4,11.2 v94.85,11.2 v102.3,11.2 | v13.3,10.95 13.3,11.2 | v30.75,41.85 36.15,36.45 39,36.45 v40.45,35 | v39.95,12.3 39.95,11.15
COL4  (via drill 0.4, 0.5)
  Top 0.254: U$69.IN arc-90 U$69.IN v9.6,4.35 | v98.55,4.35 v98.56,4.35 U$81.IN | U$67.IN 113.4,7.25 v113.4,7.7 | U$79.IN 87.4,3.91 v87.4,4.35 | U$77.IN 76.3,3.9 v76.3,4.35 | U$76.IN 64.1,4 v64.1,4.35 | U$75.IN 53.95,4.01 v54.15,4.35 | U$73.IN 44,4.07 v44.2,4.35 | U$72.IN 31.65,4.07 v31.85,4.35 | U$70.IN 20.65,3.95 v20.65,4.35 | U$2.33 29.4,46.25 v33.65,42 | v53.85,34.15 53.85,9.55 v57.3,6.1
  Bottom 0.254: v9.6,4.35 v20.65,4.35 v31.85,4.35 | 57.4,4.35 v54.15,4.35 v44.2,4.35 44.2,7.85 42.65,9.4 32.95,9.4 31.85,8.3 v31.85,4.35 | 57.4,4.35 v64.1,4.35 64.1,7.8 65.85,9.55 74.6,9.55 76.3,7.85 v76.3,4.35 87.35,4.3 v87.4,4.35 87.4,8.2 88.85,9.65 97.2,9.65 98.55,8.3 v98.55,4.35 110.05,4.35 v113.4,7.7 | v31.85,4.35 31.8,4.35 | v33.65,42 37.45,38.2 49.85,38.2 v53.85,34.15 | v57.3,6.1 57.3,4.45 57.4,4.35
DRAIN
  Top 0.61: R20.1 U$78.P$1
  Top 0.813: Q1.3 94.5,49.75 94.6,49.65
  Top 1.016: R11.1 R12.1 R13.1 R14.1 15.1 94.6,49.65 R16.1 R17.1 R19.1 R18.1 R20.1
GND  (via drill 0.5)
  Top 0.406: U$2.VIA5 21.9,48.15 U$2.THERMAL
  other vias: 3.2,39.7 119.6,41.1 120.75,1.4 2.1,1.45 16.5,47.85 106.9,21.75 74.3,47.3 73.55,52.95 79.25,58 114.65,58.55 8.25,58.6 96.6,51.2 96.75,53.2 92.65,51.1 73.8,57.95
  pour Top: 0,0 35.09,0 arc90 36.5,1.41 36.5,4 34.05,6.45 34.05,7.5 41.5,7.5 41.5,6.5 39,4 39,1.5 arc90 40.5,0 66.9,0 arc90 68.5,1.6 68.5,4 66.05,6.5 66.15,7.45 73.5,7.5 73.5,6.5 71,4 70.97,1.56 arc91 72.51,0 90.35,0 arc90 91.85,1.5 91.85,4.05 89.4,6.5 89.4,7.45 96.85,7.45 96.85,6.55 94.35,4.05 94.35,1.35 arc90 95.75,-0.05 123,0 123,2 arc90 122,3 120.05,3 arc-90 119,4.05 119,6 arc-90 120,7 122,7 arc90 123,8 123,45.3 119.72,45.27 arc-90 113.55,51.42 113.55,51.55 arc-90 119.75,57.75 119.85,57.75 123,57.7 123,61 110.8,61 76.45,61 59.55,61 0,61 0,57.74 3.29,57.74 3.25,57.75 arc-90 9.45,51.55 9.45,51.34 arc-90 3.36,45.24 0,45.3 0,8 arc90 1,7 3,7 arc-90 4.05,5.95 4.05,4.05 arc-90 3,3 1,3 arc90 0,2
  pour Bottom (rank 3): 0,0 35.09,0 arc90 36.5,1.41 36.5,4 34,6.5 34,7.5 41.5,7.5 41.5,6.5 39,4 39,1.55 arc90 40.55,0 66.99,0 arc90 68.5,1.51 68.5,4 66.05,6.5 66.1,7.5 73.5,7.45 73.5,6.5 71,4 70.97,1.58 arc91 72.53,0 90.25,0 arc90 91.85,1.6 91.85,4 89.4,6.45 89.4,7.5 96.85,7.5 96.85,6.55 94.35,4.05 94.35,1.46 arc90 95.86,-0.05 123,0 123,2 arc90 122,3 120.2,3 arc-90 119,4.2 119,6 arc-90 120,7 122,7 arc90 123,8 123,45.3 119.75,45.25 arc-180 119.75,57.75 123,57.75 123,61 109.5,61 75.85,61 0,61 0,57.75 3.25,57.75 arc-178 3.45,45.25 3.38,45.24 0,45.3 0,8 arc90 1,7 3,7 arc-90 4.05,5.95 4.05,4.05 arc-90 3,3 1,3 arc90 0,2
INT18  (via drill 0.5)
  Top 0.254: v15.8,50.1 16.65,49.25 U$2.12 | v49.25,50.9 51.45,50.9 51.45,53.05 Q2.2
  Top 0.305: 51.45,50.9 U$7.P$2
  Bottom 0.254: v15.8,50.1 25.3,50.1 27.25,52.05 48.1,52.05 v49.25,50.9
LED_GROUND0
  Top 0.254: R_LED0.2 10.5,38.1 4.85,32.45 4.85,29.55 6.52,27.88 LED11.2
LED_GROUND1  (via drill 0.5)
  Top 0.254: R_LED1.2 13.05,38.9 v13.45,38.5 | LED12.2 26.87,3.25 25.8,3.25 22.6,6.45 22.6,7.85 23.9,9.15 23.9,12.05 22.75,13.2 22.75,15.15 23.95,16.3 23.95,25.7 22.45,27.2 22.45,29.7 23.9,31.15 23.9,33.9 v24.2,34.2
  Bottom 0.254: v13.45,38.5 17.75,34.2 v24.2,34.2
LED_GROUND2
  Top 0.254: LED13.2 5,3.25 5.65,3.9 5.65,6.15 3.85,7.95 2.55,7.95 1.9,8.6 1.9,33.05 7.7,38.85 R_LED2.2
N$1  (via drill 0.5)
  Top 0.254: R11.2 82.3,46.45 v80,46.45 | v61.45,34.05 v61.45,31.6 | v25.9,27.8 LED1.2
  Bottom 0.254: v61.45,31.6 29.7,31.6 v25.9,27.8 | v61.45,34.05 62.9,35.5 69.05,35.5 v80,46.45
N$2  (via drill 0.5)
  Top 0.254: R12.2 83.05,44.8 v81.55,44.8 | v68.85,34.25 68.85,31.85 v68.7,31.7 | v45.1,28.8 45.6,27.8 LED2.2
  Bottom 0.254: v68.7,31.7 67.4,30.4 46.6,30.4 v45.1,28.8 | v81.55,44.8 71,34.25 v68.85,34.25
N$3  (via drill 0.5)
  Top 0.254: R13.2 83.1,42.5 v82.4,42.5 | v74.1,28.6 74.1,29.55 76,31.45 76,33.65 v75.05,34.6 | v63.25,28.05 61.95,26.75 61.95,23.3 62.3,22.95 62.3,21.4 61.9,21 LED3.2
  Bottom 0.254: v74.1,28.6 63.8,28.6 v63.25,28.05 | v75.05,34.6 75.05,35.15 v82.4,42.5
N$4  (via drill 0.5)
  Top 0.254: R14.2 88.1,45.1 v88.1,45.05 | v76.95,34.35 76.95,30.85 77.75,30.05 77.75,28.55 77.2,27.9 76.7,27.9 LED4.2
  Bottom 0.254: v88.1,45.05 83.8,40.75 v76.95,34.35
N$6  (via drill 0.5)
  Top 0.254: v90.95,16.55 v90.95,34.3 | v90.75,44.85 93.4,47.5 15.2 | v25.55,14.2 25,13.65 LED5.2
  Bottom 0.254: v25.55,14.2 27.45,16.2 90.6,16.2 v90.95,16.55 | v90.95,34.3 90.95,44.65 v90.75,44.85
N$7  (via drill 0.5)
  Top 0.254: LED6.2 47.2,13.5 v48.15,14.4 | v93.65,44.8 95.8,46.95 R16.2 | v100.3,14.35 100.3,15.7 99.55,16.45 99.55,18.75 100.9,20.1 100.9,21.85 99.6,23.15 99.6,25.65 100.9,26.95 100.9,30.05 99.2,31.7 99.2,34.4 v99.55,34.7
  Bottom 0.254: v48.15,14.4 48.75,15 93.15,15 94.15,16 98.65,16 v100.3,14.35 | v93.65,44.8 93.65,36.05 95.75,33.9 98.65,33.9 v99.55,34.7
N$8  (via drill 0.5)
  Top 0.254: v117.8,13 117.8,36.6 v111.1,43.3 | v98.3,44.7 R17.2 | LED7.2 61.25,7.55 61.95,8.1 61.95,12.5 v63.1,13.65
  Bottom 0.254: v63.1,13.65 63.75,13 v117.8,13 | v111.1,43.3 109.7,44.7 v98.3,44.7
N$9  (via drill 0.6)
  Top 0.254: R18.2 103.05,44.3 108.55,38.8 108.55,28.05 v107.95,27.45 | v98.7,26.85 LED8.2
  Bottom 0.254: v107.95,27.45 99.3,27.45 v98.7,26.85
N$10  (via drill 0.5)
  Top 0.254: R19.2 100.75,43.95 v102.05,42.65 | v78.2,14.05 77.55,13.4 LED9.2 | v98,35 98,31.6 96.15,29.75 96.15,27.2 97.75,25.6 97.75,23.15 96.35,21.75 96.35,20.3 97.6,19.05 97.6,16.45 96.45,15.3 96.45,14.45 96.25,14.25 v95.95,14.25
  Bottom 0.254: v102.05,42.65 102.05,39.2 v98,35 | v95.95,14.25 78.4,14.25 v78.2,14.05
N$11  (via drill 0.6)
  Top 0.254: R20.2 105.6,45.15 109.9,40.85 109.9,11.85 v109.05,11 | v101,6.95 98.65,9.3 LED10.2
  Bottom 0.254: v109.05,11 105,6.95 v101,6.95
N$13
  Top 0.406: Q2.1 PNP_UP.2 PNP_DOWN.1
N$14  (via drill 0.5)
  Top 0.254: 22.07,56.58 21.3,57.35 18.75,57.35 14.35,52.95 14.35,48.7 15.2,47.85 v15.2,42.35 | 22.07,56.58 22.15,56.5 U$2.7 | v18.25,36.25 15.25,33.25 15.25,27.65 16.75,26.15 16.75,20.85 16.7,18.75 16.7,8.7 v18.1,7.3 | 26.93,4.55 LED12.1 26.9,5.45 v28,6.55 | U$71.P$1 26.85,54.95 25.2,56.6 25.2,57.65 24.65,58.2 23.7,58.2 22.07,56.58
  Bottom 0.254: v15.2,42.35 18.25,39.3 v18.25,36.25 | v18.1,7.3 27.25,7.3 v28,6.55
N$15  (via drill 0.5, 0.6)
  Top 0.254: U$2.6 22.65,54.4 | 22.65,54.4 22.65,55.7 v24.25,57.3 | U$53.P$1 24.25,54.4 22.65,54.4 | v6.05,31.3 7.2,30.15 LED11.1
  Bottom 0.254: v24.25,57.3 23.1,58.45 17.2,58.45 12.55,53.8 12.55,48.9 10.3,46.65 10.3,37.65 6.05,33.4 v6.05,31.3
N$16  (via drill 0.5)
  Top 0.254: v13.15,46.75 10.95,44.55 6.65,44.55 5,42.9 5,36.8 1.45,33.25 1.45,8.25 2.2,7.5 3.7,7.5 4.85,6.35 LED13.1 | v18.75,55.95 19.7,56.9 21.1,56.9 21.65,56.35 U$2.8 | U$74.P$1 29.25,54.5 29.25,52.65 28.8,52.2 v25.55,52.2
  Bottom 0.254: v13.15,46.75 14,47.6 14,51.55 15.28,52.83 | 15.28,52.83 18.4,55.95 v18.75,55.95 | v25.55,52.2 25,51.65 16.6,51.65 15.43,52.83 15.28,52.83
N$17
  Top 0.254: PNP_DOWN1.2 32.55,52.25 32.55,54.25 33.3,55 U$1.1
ROW0
  Top 0.254: U$69.OUT 6.8,8.58 6.8,8.9 7.75,9.85 7.75,11.65 6.79,12.61 U$54.OUT 5.9,15.65 5.85,15.65 arc-90 4,17.5 4,17.54 arc-90 U$39.OUT 5.9,22.45 5.85,22.45 arc-90 3.9,24.4 arc-94 U$24.OUT 8.84,26.29 9.5,26.95 9.5,30.4 9.15,30.75 8.7,30.75 7.71,31.74 U$9.OUT 7.71,33.46 8.85,34.6 13.75,34.6 17.2,38.05 17.2,46.3 18.65,47.75 U$2.15
ROW1
  Top 0.254: U$68.OUT 13.3,12.41 13.3,22.45 13.1,22.45 arc-90 11.35,24.2 11.35,24.32 arc-90 U$38.OUT 13.32,33.47 17.65,37.8 17.65,46.1 18.8,47.25 U$2.16
ROW2
  Top 0.254: U$70.OUT 20.73,8.73 arc-90 20.75,8.75 20.65,8.75 arc-90 18.75,10.65 arc-91 U$55.OUT arc-90 20.7,12.64 20.7,15.7 arc-90 18.7,17.7 18.7,17.95 arc-90 20.2,19.45 U$40.OUT arc-90 20.65,19.53 20.65,22.45 arc-90 18.75,24.35 18.75,24.65 arc-90 20.39,26.29 U$25.OUT arc-90 20.7,26.32 20.7,30.65 arc-90 18.85,32.5 18.85,33.1 arc-90 20.28,34.53 U$11.OUT 20.73,37.32 18.1,39.95 18.1,45.95 18.9,46.75 U$2.17
ROW3
  Top 0.254: U$72.OUT 28.95,8.67 28.95,8.95 29.9,9.9 29.9,11.9 29.19,12.61 U$56.OUT arc-90 28.1,12.65 28.1,15.6 arc-90 26.2,17.5 26.2,17.8 arc-90 27.85,19.45 U$41.OUT arc-90 28.1,19.49 28.1,22.5 arc-90 26.15,24.45 26.15,24.55 arc-90 27.89,26.29 U$26.OUT arc-90 28.1,26.33 28.1,30.75 arc-90 26.25,32.6 26.25,32.75 arc-90 28.03,34.53 U$12.OUT 27.27,35.4 23.4,35.4 18.6,40.2 18.6,45.8 19.05,46.25 U$2.18
ROW4
  Top 0.254: U$57.OUT 35.55,15.65 arc-90 33.65,17.55 33.65,17.7 arc-90 35.4,19.45 U$42.OUT 35.56,22.44 35.5,22.5 arc-90 33.6,24.4 33.6,24.65 arc-90 35.24,26.29 U$27.OUT arc-90 35.5,26.35 35.5,30.8 arc-90 33.5,32.8 33.5,33.05 arc-90 34.98,34.53 U$13.OUT 34.24,35.85 23.65,35.85 19.1,40.4 19.1,45.55 19.3,45.75 U$2.19
ROW5
  Top 0.254: U$73.OUT 43,6.97 43,8.75 arc90 44.9,10.65 44.9,10.8 arc90 43.09,12.61 U$58.OUT 42.97,15.85 41.8,15.85 arc-90 41.3,16.35 41.3,18.35 arc-90 42.4,19.45 U$43.OUT arc-90 42.95,19.47 42.95,22.45 arc-90 40.9,24.5 40.9,24.65 arc-90 42.54,26.29 U$28.OUT arc90 43,26.32 43,30.7 arc-90 41,32.7 41,32.8 arc-90 42.73,34.53 U$14.OUT 41.2,36.3 23.9,36.3 19.9,40.3 U$2.20 19.85,45.25
ROW6
  Top 0.254: U$75.OUT 51.65,9.2 52.15,9.7 52.15,11.8 51.34,12.61 U$59.OUT arc90 50.4,12.63 50.4,15.7 50.2,15.7 arc-90 48.35,17.55 arc-94 U$44.OUT arc-90 50.35,19.48 50.35,22.45 arc-90 48.35,24.45 48.35,24.85 arc-90 49.79,26.29 U$29.OUT arc90 50.4,26.31 50.4,30.65 arc-90 48.5,32.55 48.5,32.9 arc-90 50.13,34.53 U$15.OUT 49.51,35.4 42.75,35.4 41.4,36.75 24.1,36.75 20.65,40.2 U$2.21
ROW7
  Top 0.254: U$60.OUT 57.8,15.7 arc-90 55.8,17.7 arc-90 57.55,19.45 U$45.OUT arc-90 57.75,19.49 57.75,22.45 arc-90 55.9,24.3 55.9,24.6 arc-90 57.59,26.29 U$30.OUT arc90 U$30.OUT 57.8,30.65 arc-90 55.9,32.55 55.9,32.85 arc-90 57.58,34.53 U$16.OUT 56.97,35.35 50.2,35.35 49.7,35.85 42.95,35.85 41.6,37.2 24.3,37.2 21.15,40.35 U$2.22
ROW8
  Top 0.254: U$76.OUT 64.25,6.05 64.25,9.1 63.3,10.05 63.3,11.45 64.46,12.61 U$61.OUT arc-90 U$61.OUT 65.2,15.65 65,15.65 arc-90 63.15,17.5 arc-93 U$46.OUT arc-90 U$46.OUT 65.2,22.5 arc-90 63.25,24.45 63.25,24.8 arc-90 64.74,26.29 U$31.OUT arc-90 U$31.OUT 65.2,30.75 arc-90 63.3,32.65 63.3,33.1 arc-90 64.73,34.53 U$17.OUT 64.64,35.1 59.25,35.1 58.55,35.8 50.35,35.8 49.85,36.3 43.1,36.3 41.75,37.65 24.5,37.65 21.65,40.5 U$2.23
ROW9
  Top 0.254: U$2.24 22.15,40.65 24.7,38.1 41.95,38.1 43.3,36.75 50,36.75 50.5,36.25 58.8,36.25 59.5,35.55 69.3,35.55 70.32,34.53 U$18.OUT 72.38,34.53 arc90 70.75,32.9 70.75,32.65 arc90 72.7,30.7 72.7,26.32 arc-90 U$32.OUT 72.96,26.29 arc-90 74.6,24.65 74.6,24.5 arc-90 72.65,22.55 72.65,19.47 arc90 U$47.OUT 73,19.45 arc-90 74.5,17.95 74.5,16.7 arc-90 73.55,15.75 72.67,15.75 U$62.OUT 73.69,12.61 74.45,11.85 74.45,10 73.4,8.95 73.4,8.7 75.15,8.7 76.3,7.55 76.3,5.8 U$77.OUT
ROW10
  Top 0.254: U$63.OUT arc90 80.05,12.63 80.05,15.6 arc-90 78.15,17.5 78.15,17.57 arc-90 U$48.OUT arc90 80.05,19.47 80.05,22.45 arc-90 78.05,24.45 78.05,24.6 arc-90 79.74,26.29 U$33.OUT arc90 80.05,26.31 80.05,30.7 arc-90 78.15,32.6 78.15,32.8 arc-90 79.88,34.53 U$19.OUT | U$2.25 22.65,40.8 24.9,38.55 42.15,38.55 43.5,37.2 50.15,37.2 50.65,36.7 58.95,36.7 59.65,36 69.5,36 70.15,35.35 79.21,35.35 U$19.OUT | 79.5,34.85 79.71,34.85 U$19.OUT
ROW11
  Top 0.254: U$79.OUT 87.44,8.95 86.55,8.95 arc-90 85.6,9.9 85.6,11.25 arc-90 86.96,12.61 U$64.OUT 87.44,15.59 arc-90 87.45,15.6 arc91 89.35,17.55 arc87 U$49.OUT arc90 U$49.OUT 87.45,22.4 arc-90 85.5,24.35 85.5,24.65 arc-90 87.14,26.29 U$34.OUT arc90 U$34.OUT 87.45,30.7 arc-90 85.65,32.5 85.65,33 arc-90 87.18,34.53 U$20.OUT 86.52,35.45 79.75,35.45 79.4,35.8 70.3,35.8 69.65,36.45 59.8,36.45 59.1,37.15 50.8,37.15 50.3,37.65 43.65,37.65 42.3,39 25.1,39 23.15,40.95 U$2.26
ROW12
  Top 0.254: U$2.27 23.65,41.1 25.3,39.45 42.5,39.45 43.85,38.1 50.45,38.1 50.95,37.6 59.25,37.6 60,36.85 69.85,36.85 70.5,36.2 79.6,36.2 79.9,35.9 86.7,35.9 87.15,35.45 93.94,35.45 U$21.OUT 95.12,34.53 arc-90 96.75,32.9 96.75,32.6 arc-90 94.85,30.7 U$35.OUT arc90 U$35.OUT 95.16,26.29 arc-90 96.75,24.7 96.75,24.3 arc-90 94.85,22.4 U$50.OUT arc90 U$50.OUT arc96 92.8,17.6 arc90 94.7,15.7 94.85,15.7 U$65.OUT 95.74,12.61 96.75,11.6 96.75,10 96,9 97.3,9 98.5,7.8 98.5,5.83 U$81.OUT
ROW13
  Top 0.254: U$66.OUT 102.25,15.65 arc-90 100.3,17.6 100.3,17.65 arc-90 102.1,19.45 U$51.OUT arc-90 102.25,19.47 102.25,22.45 arc90 104.15,24.35 104.15,24.8 arc90 102.66,26.29 U$36.OUT arc-90 102.25,26.31 102.25,30.7 arc-90 100.45,32.5 100.45,32.95 arc-90 102.03,34.53 U$22.OUT 100.95,35.85 87.35,35.85 86.85,36.35 80.05,36.35 79.75,36.65 70.65,36.65 70,37.3 60.15,37.3 59.4,38.05 51.1,38.05 50.6,38.55 44,38.55 42.6,39.95 25.45,39.95 24.15,41.25 U$2.28
ROW14  (via drill 0.5)
  Top 0.254: U$23.OUT 114.22,34.53 arc-90 115.2,32.8 115.2,32.5 arc-90 113.4,30.7 U$37.OUT arc-90 U$37.OUT 113.76,26.29 arc-90 115.35,24.7 115.35,24.35 arc-90 113.4,22.4 U$52.OUT arc-90 U$52.OUT 113.9,19.35 arc-90 115.15,18.1 115.4,17.6 arc-90 113.4,15.6 113.4,9.16 arc-90 U$67.OUT 109,9.15 105.1,13.05 105.1,15.85 105.75,16.5 105.75,34.1 103.55,36.3 87.55,36.3 87.05,36.8 80.2,36.8 79.9,37.1 70.85,37.1 70.2,37.75 60.3,37.75 59.55,38.5 51.25,38.5 50.75,39 45.15,39 v41.7,42.45 | U$2.40 27.95,49.75 v28.7,50.5
  Bottom 0.254: v28.7,50.5 34.95,50.5 41.7,43.75 v41.7,42.45
SCL18  (via drill 0.4, 0.5)
  Top 0.254: v18.2,53.65 18.2,50 18.45,49.75 U$2.11 | U$1.6 40.45,54 v40.9,54.55
  Top 0.305: v63.4,47.95 63.4,45.7 U$6.P$2
  Bottom 0.254: v63.4,47.95 56.8,54.55 v40.9,54.55 19.1,54.55 v18.2,53.65
  Bottom 0.305: 63.4,45.7 U$6.P$2
SDA18  (via drill 0.4, 0.5)
  Top 0.254: v19.9,53.25 20.65,52.5 U$2.10 | U$1.5 38,53.45 v43.75,53.45
  Top 0.305: v59.4,47.9 59.4,45.7 U$5.P$2
  Bottom 0.254: v43.75,53.45 53.85,53.45 v59.4,47.9 | v43.75,53.45 43,53.45 | v19.9,53.25 20.1,53.45 v43.75,53.45
  Bottom 0.305: 59.4,45.7 U$5.P$2
VCC
  Top 0.254: 32.23,48.98 32.15,49 | U$1.8 36.55,56.4 31.95,56.4 31.4,55.85 31.4,53.5 30.45,52.55 30.45,49 | PNP_DOWN1.1 32.25,50.27 32.23,50.25 | U$2.39 26.9,49.25 27.15,49 26.9,48.75 U$2.38 | 34.2,49 C3.1
  Top 0.406: 32.23,50.25 32.23,48.98
  Top 0.61: 30.6,49 27.15,49
  Top 0.813: C3.1 34.9,49.7 VOLTAGE_REGULATOR.2 | 34.2,49 32.15,49 30.6,49 30.45,49

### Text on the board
tPlace: R4 | C3 | MOSFET | R1 | R2 | R3
tNames: _ | + | connection / detector | INT | _ | EEPROM | backlight | R5-R14 | C1 | C2 | PNP | + | MCP1700 | 1 | 2 | 3 | 4 | 5 | 6 | 7 | 8 | 9 | 10 | TOHKBD_2.0.6.6 / by Dirk van Leersum | matrix controller | 1 | 4 | 9 | 2 | 3 | 7 | 5 | 6 | 8 | 10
